DATA_BLOCK DB 3


STRUCT
    D_0 : word := W#16#0;
    D_1 : word := W#16#0;
    D_2 : word := W#16#0;
    D_3 : word := W#16#0;
    D_4 : word := W#16#0;
    D_5 : word := W#16#0;
    D_6 : word := W#16#0;
    D_7 : word := W#16#0;
    D_8 : word := W#16#0;
    D_9 : word := W#16#3;
    D_10 : word := W#16#0;
    D_11 : word := W#16#200;
    D_12 : word := W#16#0;
    D_13 : word := W#16#4000;
    D_14 : word := W#16#0;
    D_15 : word := W#16#4000;
    D_16 : word := W#16#0;
    D_17 : word := W#16#200;
    D_18 : word := W#16#0;
    D_19 : word := W#16#200;
    D_20 : word := W#16#0;
    D_21 : word := W#16#200;
    D_22 : word := W#16#0;
    D_23 : word := W#16#200;
    D_24 : word := W#16#0;
    D_25 : word := W#16#200;
    D_26 : word := W#16#0;
    D_27 : word := W#16#200;
    D_28 : word := W#16#0;
    D_29 : word := W#16#200;
    D_30 : word := W#16#0;
    D_31 : word := W#16#200;
    D_32 : word := W#16#0;
  END_STRUCT
BEGIN

END_DATA_BLOCK

DATA_BLOCK DB 9


STRUCT
    D_0 : word := W#16#0;
    D_1 : word := W#16#0;
    D_2 : word := W#16#0;
    D_3 : word := W#16#0;
    D_4 : word := W#16#0;
    D_5 : word := W#16#0;
    D_6 : word := W#16#0;
    D_7 : word := W#16#0;
    D_8 : word := W#16#0;
    D_9 : word := W#16#0;
    D_10 : word := W#16#508;
    D_11 : word := W#16#2C00;
    D_12 : word := W#16#0;
    D_13 : word := W#16#F;
    D_14 : word := W#16#112E;
    D_15 : word := W#16#0;
  END_STRUCT
BEGIN

END_DATA_BLOCK

DATA_BLOCK DB 94


STRUCT
    D_0 : word := W#16#0;
    D_1 : word := W#16#25;
    D_2 : word := W#16#12;
    D_3 : word := W#16#200;
    D_4 : word := W#16#100;
    D_5 : word := W#16#100;
    D_6 : word := W#16#78;
    D_7 : word := W#16#3018;
    D_8 : word := W#16#2060;
    D_9 : word := W#16#0;
    D_10 : word := W#16#0;
    D_11 : word := W#16#0;
    D_12 : word := W#16#0;
    D_13 : word := W#16#0;
    D_14 : word := W#16#0;
    D_15 : word := W#16#0;
    D_16 : word := W#16#0;
    D_17 : word := W#16#2010;
    D_18 : word := W#16#2030;
    D_19 : word := W#16#2010;
    D_20 : word := W#16#1050;
    D_21 : word := W#16#2020;
    D_22 : word := W#16#2020;
    D_23 : word := W#16#2010;
    D_24 : word := W#16#2060;
    D_25 : word := W#16#2300;
    D_26 : word := W#16#2010;
    D_27 : word := W#16#2020;
    D_28 : word := W#16#2005;
    D_29 : word := W#16#2030;
    D_30 : word := W#16#2008;
    D_31 : word := W#16#2300;
    D_32 : word := W#16#1020;
    D_33 : word := W#16#1020;
    D_34 : word := W#16#2008;
    D_35 : word := W#16#2300;
    D_36 : word := W#16#2008;
    D_37 : word := W#16#2025;
    D_38 : word := W#16#2015;
    D_39 : word := W#16#2015;
    D_40 : word := W#16#2300;
    D_41 : word := W#16#1050;
    D_42 : word := W#16#1050;
    D_43 : word := W#16#1050;
    D_44 : word := W#16#2020;
    D_45 : word := W#16#2008;
    D_46 : word := W#16#2300;
    D_47 : word := W#16#2010;
    D_48 : word := W#16#2300;
    D_49 : word := W#16#2030;
    D_50 : word := W#16#2010;
    D_51 : word := W#16#2030;
    D_52 : word := W#16#2010;
    D_53 : word := W#16#2030;
    D_54 : word := W#16#1020;
    D_55 : word := W#16#1020;
    D_56 : word := W#16#1020;
    D_57 : word := W#16#1020;
    D_58 : word := W#16#1020;
    D_59 : word := W#16#1020;
    D_60 : word := W#16#3180;
    D_61 : word := W#16#2300;
    D_62 : word := W#16#2300;
    D_63 : word := W#16#1050;
    D_64 : word := W#16#1150;
    D_65 : word := W#16#2010;
    D_66 : word := W#16#2002;
    D_67 : word := W#16#2002;
    D_68 : word := W#16#2002;
    D_69 : word := W#16#2030;
    D_70 : word := W#16#2030;
    D_71 : word := W#16#2020;
    D_72 : word := W#16#2020;
    D_73 : word := W#16#2020;
    D_74 : word := W#16#2045;
    D_75 : word := W#16#2030;
    D_76 : word := W#16#2030;
    D_77 : word := W#16#2005;
    D_78 : word := W#16#2005;
    D_79 : word := W#16#2005;
    D_80 : word := W#16#2005;
    D_81 : word := W#16#2120;
    D_82 : word := W#16#2010;
    D_83 : word := W#16#2010;
    D_84 : word := W#16#2009;
    D_85 : word := W#16#2005;
    D_86 : word := W#16#2005;
    D_87 : word := W#16#2010;
    D_88 : word := W#16#2300;
    D_89 : word := W#16#0;
    D_90 : word := W#16#2180;
    D_91 : word := W#16#2180;
    D_92 : word := W#16#3030;
    D_93 : word := W#16#2015;
    D_94 : word := W#16#2120;
    D_95 : word := W#16#2300;
    D_96 : word := W#16#2420;
    D_97 : word := W#16#2420;
    D_98 : word := W#16#2300;
    D_99 : word := W#16#1010;
    D_100 : word := W#16#1010;
    D_101 : word := W#16#2060;
    D_102 : word := W#16#2300;
    D_103 : word := W#16#2060;
    D_104 : word := W#16#1020;
    D_105 : word := W#16#1020;
    D_106 : word := W#16#1010;
    D_107 : word := W#16#2060;
    D_108 : word := W#16#2045;
    D_109 : word := W#16#0;
    D_110 : word := W#16#0;
    D_111 : word := W#16#1010;
    D_112 : word := W#16#1020;
    D_113 : word := W#16#0;
    D_114 : word := W#16#0;
    D_115 : word := W#16#0;
    D_116 : word := W#16#0;
    D_117 : word := W#16#0;
    D_118 : word := W#16#0;
    D_119 : word := W#16#0;
    D_120 : word := W#16#0;
    D_121 : word := W#16#0;
    D_122 : word := W#16#0;
    D_123 : word := W#16#0;
    D_124 : word := W#16#0;
    D_125 : word := W#16#0;
    D_126 : word := W#16#0;
    D_127 : word := W#16#0;
    D_128 : word := W#16#0;
    D_129 : word := W#16#2002;
    D_130 : word := W#16#2003;
    D_131 : word := W#16#0;
    D_132 : word := W#16#0;
    D_133 : word := W#16#0;
  END_STRUCT
BEGIN

END_DATA_BLOCK

DATA_BLOCK DB 99


STRUCT
    D_0 : word := W#16#0;
    D_1 : word := W#16#0;
    D_2 : word := W#16#3;
    D_3 : word := W#16#6;
    D_4 : word := W#16#2;
    D_5 : word := W#16#C;
    D_6 : word := W#16#6;
    D_7 : word := W#16#6;
    D_8 : word := W#16#6;
    D_9 : word := W#16#6;
    D_10 : word := W#16#6;
    D_11 : word := W#16#6;
    D_12 : word := W#16#6;
    D_13 : word := W#16#6;
    D_14 : word := W#16#6;
    D_15 : word := W#16#6;
    D_16 : word := W#16#0;
    D_17 : word := W#16#A6;
    D_18 : word := W#16#53;
    D_19 : word := W#16#1F4;
    D_20 : word := W#16#0;
  END_STRUCT
BEGIN

END_DATA_BLOCK

DATA_BLOCK DB 100


STRUCT
    D_0 : word := W#16#0;
    D_1 : word := W#16#5A;
    D_2 : word := W#16#0;
    D_3 : word := W#16#0;
    D_4 : word := W#16#0;
    D_5 : word := W#16#0;
    D_6 : word := W#16#0;
    D_7 : word := W#16#0;
    D_8 : word := W#16#0;
    D_9 : word := W#16#0;
    D_10 : word := W#16#8001;
    D_11 : word := W#16#8000;
    D_12 : word := W#16#8002;
    D_13 : word := W#16#8100;
    D_14 : word := W#16#8104;
    D_15 : word := W#16#8104;
    D_16 : word := W#16#8001;
    D_17 : word := W#16#8104;
    D_18 : word := W#16#8000;
    D_19 : word := W#16#8004;
    D_20 : word := W#16#8104;
    D_21 : word := W#16#8104;
    D_22 : word := W#16#8100;
    D_23 : word := W#16#8104;
    D_24 : word := W#16#8900;
    D_25 : word := W#16#8104;
    D_26 : word := W#16#8000;
    D_27 : word := W#16#8004;
    D_28 : word := W#16#8104;
    D_29 : word := W#16#8104;
    D_30 : word := W#16#8100;
    D_31 : word := W#16#8104;
    D_32 : word := W#16#8106;
    D_33 : word := W#16#8104;
    D_34 : word := W#16#8100;
    D_35 : word := W#16#8104;
    D_36 : word := W#16#8900;
    D_37 : word := W#16#8104;
    D_38 : word := W#16#100;
    D_39 : word := W#16#100;
    D_40 : word := W#16#100;
    D_41 : word := W#16#100;
    D_42 : word := W#16#8004;
    D_43 : word := W#16#8004;
    D_44 : word := W#16#4129;
    D_45 : word := W#16#412D;
    D_46 : word := W#16#8100;
    D_47 : word := W#16#8801;
    D_48 : word := W#16#8004;
    D_49 : word := W#16#8000;
    D_50 : word := W#16#8000;
    D_51 : word := W#16#815A;
    D_52 : word := W#16#8000;
    D_53 : word := W#16#8000;
    D_54 : word := W#16#8801;
    D_55 : word := W#16#8100;
    D_56 : word := W#16#8002;
    D_57 : word := W#16#8002;
    D_58 : word := W#16#8001;
    D_59 : word := W#16#8004;
    D_60 : word := W#16#8000;
    D_61 : word := W#16#8104;
    D_62 : word := W#16#8002;
    D_63 : word := W#16#8001;
    D_64 : word := W#16#8000;
    D_65 : word := W#16#8000;
    D_66 : word := W#16#8004;
    D_67 : word := W#16#8100;
    D_68 : word := W#16#8104;
    D_69 : word := W#16#8102;
    D_70 : word := W#16#8100;
    D_71 : word := W#16#8100;
    D_72 : word := W#16#8000;
    D_73 : word := W#16#8000;
    D_74 : word := W#16#100;
    D_75 : word := W#16#8001;
    D_76 : word := W#16#100;
    D_77 : word := W#16#8002;
    D_78 : word := W#16#8000;
    D_79 : word := W#16#8000;
    D_80 : word := W#16#100;
    D_81 : word := W#16#8002;
    D_82 : word := W#16#8100;
    D_83 : word := W#16#8002;
    D_84 : word := W#16#8801;
    D_85 : word := W#16#8102;
    D_86 : word := W#16#8002;
    D_87 : word := W#16#8002;
    D_88 : word := W#16#8000;
    D_89 : word := W#16#8801;
    D_90 : word := W#16#100;
    D_91 : word := W#16#100;
    D_92 : word := W#16#100;
    D_93 : word := W#16#100;
    D_94 : word := W#16#100;
    D_95 : word := W#16#100;
    D_96 : word := W#16#100;
    D_97 : word := W#16#100;
    D_98 : word := W#16#100;
    D_99 : word := W#16#100;
    D_100 : word := W#16#0;
    D_101 : word := W#16#0;
    D_102 : word := W#16#0;
    D_103 : word := W#16#0;
    D_104 : word := W#16#0;
    D_105 : word := W#16#0;
    D_106 : word := W#16#0;
    D_107 : word := W#16#0;
    D_108 : word := W#16#0;
    D_109 : word := W#16#0;
    D_110 : word := W#16#F;
    D_111 : word := W#16#5;
    D_112 : word := W#16#5;
    D_113 : word := W#16#5;
    D_114 : word := W#16#5;
    D_115 : word := W#16#5;
    D_116 : word := W#16#F;
    D_117 : word := W#16#5;
    D_118 : word := W#16#5;
    D_119 : word := W#16#5;
    D_120 : word := W#16#5;
    D_121 : word := W#16#5;
    D_122 : word := W#16#5;
    D_123 : word := W#16#5;
    D_124 : word := W#16#5;
    D_125 : word := W#16#5;
    D_126 : word := W#16#5;
    D_127 : word := W#16#5;
    D_128 : word := W#16#5;
    D_129 : word := W#16#5;
    D_130 : word := W#16#5;
    D_131 : word := W#16#5;
    D_132 : word := W#16#5;
    D_133 : word := W#16#5;
    D_134 : word := W#16#5;
    D_135 : word := W#16#5;
    D_136 : word := W#16#5;
    D_137 : word := W#16#5;
    D_138 : word := W#16#5;
    D_139 : word := W#16#5;
    D_140 : word := W#16#5;
    D_141 : word := W#16#5;
    D_142 : word := W#16#5;
    D_143 : word := W#16#5;
    D_144 : word := W#16#0;
    D_145 : word := W#16#0;
    D_146 : word := W#16#5;
    D_147 : word := W#16#F;
    D_148 : word := W#16#5;
    D_149 : word := W#16#5;
    D_150 : word := W#16#5;
    D_151 : word := W#16#5;
    D_152 : word := W#16#5;
    D_153 : word := W#16#5;
    D_154 : word := W#16#F;
    D_155 : word := W#16#5;
    D_156 : word := W#16#5;
    D_157 : word := W#16#5;
    D_158 : word := W#16#F;
    D_159 : word := W#16#5;
    D_160 : word := W#16#5;
    D_161 : word := W#16#5;
    D_162 : word := W#16#5;
    D_163 : word := W#16#F;
    D_164 : word := W#16#5;
    D_165 : word := W#16#5;
    D_166 : word := W#16#5;
    D_167 : word := W#16#5;
    D_168 : word := W#16#5;
    D_169 : word := W#16#5;
    D_170 : word := W#16#5;
    D_171 : word := W#16#5;
    D_172 : word := W#16#5;
    D_173 : word := W#16#5;
    D_174 : word := W#16#5;
    D_175 : word := W#16#F;
    D_176 : word := W#16#5;
    D_177 : word := W#16#5;
    D_178 : word := W#16#5;
    D_179 : word := W#16#F;
    D_180 : word := W#16#5;
    D_181 : word := W#16#5;
    D_182 : word := W#16#5;
    D_183 : word := W#16#5;
    D_184 : word := W#16#F;
    D_185 : word := W#16#5;
    D_186 : word := W#16#5;
    D_187 : word := W#16#5;
    D_188 : word := W#16#5;
    D_189 : word := W#16#F;
    D_190 : word := W#16#5;
    D_191 : word := W#16#5;
    D_192 : word := W#16#5;
    D_193 : word := W#16#5;
    D_194 : word := W#16#5;
    D_195 : word := W#16#5;
    D_196 : word := W#16#5;
    D_197 : word := W#16#5;
    D_198 : word := W#16#5;
    D_199 : word := W#16#5;
    D_200 : word := W#16#0;
  END_STRUCT
BEGIN

END_DATA_BLOCK

DATA_BLOCK DB 108


STRUCT
    D_0 : word := W#16#0;
    D_1 : word := W#16#0;
    D_2 : word := W#16#0;
    D_3 : word := W#16#0;
    D_4 : word := W#16#0;
    D_5 : word := W#16#0;
    D_6 : word := W#16#0;
    D_7 : word := W#16#0;
    D_8 : word := W#16#0;
    D_9 : word := W#16#0;
    D_10 : word := W#16#300;
    D_11 : word := W#16#3;
    D_12 : word := W#16#404;
    D_13 : word := W#16#300;
    D_14 : word := W#16#303;
    D_15 : word := W#16#404;
    D_16 : word := W#16#400;
    D_17 : word := W#16#303;
    D_18 : word := W#16#303;
    D_19 : word := W#16#404;
    D_20 : word := W#16#400;
    D_21 : word := W#16#406;
    D_22 : word := W#16#300;
    D_23 : word := W#16#303;
    D_24 : word := W#16#0;
    D_25 : word := W#16#0;
    D_26 : word := W#16#303;
    D_27 : word := W#16#202;
    D_28 : word := W#16#0;
    D_29 : word := W#16#303;
    D_30 : word := W#16#5A03;
    D_31 : word := W#16#303;
    D_32 : word := W#16#300;
    D_33 : word := W#16#303;
    D_34 : word := W#16#300;
    D_35 : word := W#16#303;
    D_36 : word := W#16#3;
    D_37 : word := W#16#303;
    D_38 : word := W#16#303;
    D_39 : word := W#16#303;
    D_40 : word := W#16#303;
    D_41 : word := W#16#303;
    D_42 : word := W#16#0;
    D_43 : word := W#16#300;
    D_44 : word := W#16#303;
    D_45 : word := W#16#300;
    D_46 : word := W#16#303;
    D_47 : word := W#16#300;
    D_48 : word := W#16#303;
    D_49 : word := W#16#3;
    D_50 : word := W#16#0;
    D_51 : word := W#16#0;
    D_52 : word := W#16#0;
    D_53 : word := W#16#0;
    D_54 : word := W#16#0;
    D_55 : word := W#16#0;
    D_56 : word := W#16#0;
    D_57 : word := W#16#0;
    D_58 : word := W#16#0;
    D_59 : word := W#16#0;
    D_60 : word := W#16#0;
  END_STRUCT
BEGIN

END_DATA_BLOCK

DATA_BLOCK DB 110


STRUCT
    D_0 : word := W#16#0;
    D_1 : word := W#16#3A;
    D_2 : word := W#16#0;
    D_3 : word := W#16#0;
    D_4 : word := W#16#0;
    D_5 : word := W#16#0;
    D_6 : word := W#16#0;
    D_7 : word := W#16#0;
    D_8 : word := W#16#0;
    D_9 : word := W#16#0;
    D_10 : word := W#16#8128;
    D_11 : word := W#16#8128;
    D_12 : word := W#16#8128;
    D_13 : word := W#16#8128;
    D_14 : word := W#16#404A;
    D_15 : word := W#16#484A;
    D_16 : word := W#16#102;
    D_17 : word := W#16#C828;
    D_18 : word := W#16#C128;
    D_19 : word := W#16#C128;
    D_20 : word := W#16#100;
    D_21 : word := W#16#802;
    D_22 : word := W#16#802;
    D_23 : word := W#16#C118;
    D_24 : word := W#16#101;
    D_25 : word := W#16#8128;
    D_26 : word := W#16#8128;
    D_27 : word := W#16#8128;
    D_28 : word := W#16#100;
    D_29 : word := W#16#100;
    D_30 : word := W#16#100;
    D_31 : word := W#16#100;
    D_32 : word := W#16#100;
    D_33 : word := W#16#100;
    D_34 : word := W#16#100;
    D_35 : word := W#16#100;
    D_36 : word := W#16#100;
    D_37 : word := W#16#100;
    D_38 : word := W#16#100;
    D_39 : word := W#16#100;
    D_40 : word := W#16#102;
    D_41 : word := W#16#102;
    D_42 : word := W#16#102;
    D_43 : word := W#16#102;
    D_44 : word := W#16#102;
    D_45 : word := W#16#102;
    D_46 : word := W#16#101;
    D_47 : word := W#16#102;
    D_48 : word := W#16#100;
    D_49 : word := W#16#100;
    D_50 : word := W#16#100;
    D_51 : word := W#16#100;
    D_52 : word := W#16#100;
    D_53 : word := W#16#100;
    D_54 : word := W#16#100;
    D_55 : word := W#16#100;
    D_56 : word := W#16#100;
    D_57 : word := W#16#102;
    D_58 : word := W#16#100;
    D_59 : word := W#16#100;
    D_60 : word := W#16#100;
    D_61 : word := W#16#100;
    D_62 : word := W#16#100;
    D_63 : word := W#16#100;
    D_64 : word := W#16#100;
    D_65 : word := W#16#100;
    D_66 : word := W#16#100;
    D_67 : word := W#16#100;
    D_68 : word := W#16#100;
    D_69 : word := W#16#100;
    D_70 : word := W#16#0;
    D_71 : word := W#16#0;
    D_72 : word := W#16#0;
    D_73 : word := W#16#0;
    D_74 : word := W#16#0;
    D_75 : word := W#16#0;
    D_76 : word := W#16#0;
    D_77 : word := W#16#0;
    D_78 : word := W#16#0;
    D_79 : word := W#16#0;
    D_80 : word := W#16#0;
    D_81 : word := W#16#0;
    D_82 : word := W#16#0;
    D_83 : word := W#16#0;
    D_84 : word := W#16#0;
    D_85 : word := W#16#0;
    D_86 : word := W#16#0;
    D_87 : word := W#16#0;
    D_88 : word := W#16#0;
    D_89 : word := W#16#0;
    D_90 : word := W#16#0;
    D_91 : word := W#16#0;
    D_92 : word := W#16#0;
    D_93 : word := W#16#0;
    D_94 : word := W#16#0;
    D_95 : word := W#16#0;
    D_96 : word := W#16#0;
    D_97 : word := W#16#0;
    D_98 : word := W#16#0;
    D_99 : word := W#16#0;
    D_100 : word := W#16#0;
    D_101 : word := W#16#0;
    D_102 : word := W#16#0;
    D_103 : word := W#16#0;
    D_104 : word := W#16#0;
    D_105 : word := W#16#0;
    D_106 : word := W#16#0;
    D_107 : word := W#16#0;
    D_108 : word := W#16#0;
    D_109 : word := W#16#0;
    D_110 : word := W#16#14;
    D_111 : word := W#16#14;
    D_112 : word := W#16#14;
    D_113 : word := W#16#14;
    D_114 : word := W#16#14;
    D_115 : word := W#16#14;
    D_116 : word := W#16#14;
    D_117 : word := W#16#0;
    D_118 : word := W#16#0;
    D_119 : word := W#16#0;
    D_120 : word := W#16#14;
    D_121 : word := W#16#14;
    D_122 : word := W#16#14;
    D_123 : word := W#16#0;
    D_124 : word := W#16#14;
    D_125 : word := W#16#14;
    D_126 : word := W#16#14;
    D_127 : word := W#16#14;
    D_128 : word := W#16#14;
    D_129 : word := W#16#14;
    D_130 : word := W#16#14;
    D_131 : word := W#16#14;
    D_132 : word := W#16#14;
    D_133 : word := W#16#14;
    D_134 : word := W#16#14;
    D_135 : word := W#16#14;
    D_136 : word := W#16#14;
    D_137 : word := W#16#14;
    D_138 : word := W#16#14;
    D_139 : word := W#16#14;
    D_140 : word := W#16#14;
    D_141 : word := W#16#14;
    D_142 : word := W#16#14;
    D_143 : word := W#16#14;
    D_144 : word := W#16#14;
    D_145 : word := W#16#14;
    D_146 : word := W#16#14;
    D_147 : word := W#16#14;
    D_148 : word := W#16#14;
    D_149 : word := W#16#14;
    D_150 : word := W#16#14;
    D_151 : word := W#16#14;
    D_152 : word := W#16#14;
    D_153 : word := W#16#14;
    D_154 : word := W#16#14;
    D_155 : word := W#16#14;
    D_156 : word := W#16#14;
    D_157 : word := W#16#14;
    D_158 : word := W#16#14;
    D_159 : word := W#16#14;
    D_160 : word := W#16#14;
    D_161 : word := W#16#14;
    D_162 : word := W#16#14;
    D_163 : word := W#16#14;
    D_164 : word := W#16#14;
    D_165 : word := W#16#14;
    D_166 : word := W#16#14;
    D_167 : word := W#16#14;
    D_168 : word := W#16#14;
    D_169 : word := W#16#14;
    D_170 : word := W#16#14;
    D_171 : word := W#16#14;
    D_172 : word := W#16#14;
    D_173 : word := W#16#14;
    D_174 : word := W#16#14;
    D_175 : word := W#16#14;
    D_176 : word := W#16#14;
    D_177 : word := W#16#14;
    D_178 : word := W#16#14;
    D_179 : word := W#16#14;
    D_180 : word := W#16#14;
    D_181 : word := W#16#14;
    D_182 : word := W#16#14;
    D_183 : word := W#16#14;
    D_184 : word := W#16#14;
    D_185 : word := W#16#14;
    D_186 : word := W#16#14;
    D_187 : word := W#16#14;
    D_188 : word := W#16#14;
    D_189 : word := W#16#14;
    D_190 : word := W#16#14;
    D_191 : word := W#16#14;
    D_192 : word := W#16#14;
    D_193 : word := W#16#14;
    D_194 : word := W#16#14;
    D_195 : word := W#16#14;
    D_196 : word := W#16#14;
    D_197 : word := W#16#14;
    D_198 : word := W#16#14;
    D_199 : word := W#16#14;
    D_200 : word := W#16#0;
  END_STRUCT
BEGIN

END_DATA_BLOCK

DATA_BLOCK DB 118


STRUCT
    D_0 : word := W#16#0;
    D_1 : word := W#16#0;
    D_2 : word := W#16#0;
    D_3 : word := W#16#0;
    D_4 : word := W#16#0;
    D_5 : word := W#16#0;
    D_6 : word := W#16#0;
    D_7 : word := W#16#0;
    D_8 : word := W#16#0;
    D_9 : word := W#16#0;
    D_10 : word := W#16#2828;
    D_11 : word := W#16#0;
    D_12 : word := W#16#202;
    D_13 : word := W#16#200;
    D_14 : word := W#16#202;
    D_15 : word := W#16#300;
    D_16 : word := W#16#203;
    D_17 : word := W#16#2801;
    D_18 : word := W#16#2828;
    D_19 : word := W#16#0;
    D_20 : word := W#16#0;
    D_21 : word := W#16#0;
    D_22 : word := W#16#0;
    D_23 : word := W#16#0;
    D_24 : word := W#16#0;
    D_25 : word := W#16#202;
    D_26 : word := W#16#202;
    D_27 : word := W#16#202;
    D_28 : word := W#16#205;
    D_29 : word := W#16#0;
    D_30 : word := W#16#0;
    D_31 : word := W#16#0;
    D_32 : word := W#16#0;
    D_33 : word := W#16#0;
    D_34 : word := W#16#0;
    D_35 : word := W#16#0;
    D_36 : word := W#16#0;
    D_37 : word := W#16#0;
    D_38 : word := W#16#0;
    D_39 : word := W#16#0;
    D_40 : word := W#16#0;
    D_41 : word := W#16#0;
    D_42 : word := W#16#0;
    D_43 : word := W#16#0;
    D_44 : word := W#16#0;
    D_45 : word := W#16#0;
    D_46 : word := W#16#0;
    D_47 : word := W#16#0;
    D_48 : word := W#16#0;
    D_49 : word := W#16#0;
    D_50 : word := W#16#0;
    D_51 : word := W#16#0;
    D_52 : word := W#16#0;
    D_53 : word := W#16#0;
    D_54 : word := W#16#0;
    D_55 : word := W#16#0;
    D_56 : word := W#16#0;
    D_57 : word := W#16#0;
    D_58 : word := W#16#0;
    D_59 : word := W#16#0;
    D_60 : word := W#16#0;
  END_STRUCT
BEGIN

END_DATA_BLOCK

DATA_BLOCK DB 120


STRUCT
    D_0 : word := W#16#0;
    D_1 : word := W#16#0;
    D_2 : word := W#16#0;
    D_3 : word := W#16#0;
    D_4 : word := W#16#0;
    D_5 : word := W#16#0;
    D_6 : word := W#16#0;
    D_7 : word := W#16#0;
    D_8 : word := W#16#0;
    D_9 : word := W#16#0;
    D_10 : word := W#16#5FC9;
    D_11 : word := W#16#40CF;
    D_12 : word := W#16#71D7;
    D_13 : word := W#16#80;
    D_14 : word := W#16#0;
    D_15 : word := W#16#8213;
    D_16 : word := W#16#0;
    D_17 : word := W#16#416C;
    D_18 : word := W#16#8;
    D_19 : word := W#16#2000;
    D_20 : word := W#16#C;
    D_21 : word := W#16#8018;
    D_22 : word := W#16#0;
    D_23 : word := W#16#7002;
    D_24 : word := W#16#9002;
    D_25 : word := W#16#3E14;
    D_26 : word := W#16#0;
    D_27 : word := W#16#200;
    D_28 : word := W#16#0;
    D_29 : word := W#16#4000;
    D_30 : word := W#16#0;
    D_31 : word := W#16#4000;
    D_32 : word := W#16#0;
    D_33 : word := W#16#0;
    D_34 : word := W#16#0;
    D_35 : word := W#16#0;
    D_36 : word := W#16#0;
    D_37 : word := W#16#0;
    D_38 : word := W#16#0;
    D_39 : word := W#16#0;
    D_40 : word := W#16#0;
    D_41 : word := W#16#0;
    D_42 : word := W#16#0;
    D_43 : word := W#16#0;
    D_44 : word := W#16#0;
    D_45 : word := W#16#0;
    D_46 : word := W#16#0;
    D_47 : word := W#16#0;
    D_48 : word := W#16#0;
    D_49 : word := W#16#0;
    D_50 : word := W#16#0;
    D_51 : word := W#16#0;
    D_52 : word := W#16#0;
    D_53 : word := W#16#0;
    D_54 : word := W#16#0;
    D_55 : word := W#16#0;
    D_56 : word := W#16#0;
    D_57 : word := W#16#0;
    D_58 : word := W#16#0;
    D_59 : word := W#16#0;
    D_60 : word := W#16#0;
    D_61 : word := W#16#0;
    D_62 : word := W#16#0;
    D_63 : word := W#16#0;
    D_64 : word := W#16#0;
    D_65 : word := W#16#0;
    D_66 : word := W#16#0;
    D_67 : word := W#16#0;
    D_68 : word := W#16#0;
    D_69 : word := W#16#0;
    D_70 : word := W#16#0;
    D_71 : word := W#16#0;
    D_72 : word := W#16#0;
    D_73 : word := W#16#0;
    D_74 : word := W#16#0;
    D_75 : word := W#16#0;
    D_76 : word := W#16#0;
    D_77 : word := W#16#0;
    D_78 : word := W#16#0;
    D_79 : word := W#16#0;
    D_80 : word := W#16#AA00;
    D_81 : word := W#16#0;
    D_82 : word := W#16#270;
    D_83 : word := W#16#2008;
    D_84 : word := W#16#2;
    D_85 : word := W#16#E83;
    D_86 : word := W#16#0;
    D_87 : word := W#16#8002;
    D_88 : word := W#16#1E2;
    D_89 : word := W#16#9;
    D_90 : word := W#16#600;
    D_91 : word := W#16#842E;
    D_92 : word := W#16#1801;
    D_93 : word := W#16#1800;
    D_94 : word := W#16#9B73;
    D_95 : word := W#16#0;
    D_96 : word := W#16#AA00;
    D_97 : word := W#16#0;
    D_98 : word := W#16#240C;
    D_99 : word := W#16#0;
    D_100 : word := W#16#0;
    D_101 : word := W#16#0;
    D_102 : word := W#16#0;
    D_103 : word := W#16#0;
    D_104 : word := W#16#0;
    D_105 : word := W#16#0;
    D_106 : word := W#16#0;
    D_107 : word := W#16#0;
    D_108 : word := W#16#0;
    D_109 : word := W#16#1;
    D_110 : word := W#16#1EEF;
    D_111 : word := W#16#FCFF;
    D_112 : word := W#16#FF0E;
    D_113 : word := W#16#0;
    D_114 : word := W#16#0;
    D_115 : word := W#16#0;
    D_116 : word := W#16#0;
    D_117 : word := W#16#0;
    D_118 : word := W#16#0;
    D_119 : word := W#16#0;
    D_120 : word := W#16#0;
    D_121 : word := W#16#0;
    D_122 : word := W#16#0;
    D_123 : word := W#16#0;
    D_124 : word := W#16#0;
    D_125 : word := W#16#0;
    D_126 : word := W#16#0;
    D_127 : word := W#16#0;
    D_128 : word := W#16#0;
    D_129 : word := W#16#0;
    D_130 : word := W#16#0;
    D_131 : word := W#16#0;
    D_132 : word := W#16#0;
    D_133 : word := W#16#0;
    D_134 : word := W#16#0;
    D_135 : word := W#16#0;
    D_136 : word := W#16#0;
    D_137 : word := W#16#0;
    D_138 : word := W#16#0;
    D_139 : word := W#16#0;
    D_140 : word := W#16#0;
    D_141 : word := W#16#0;
    D_142 : word := W#16#0;
    D_143 : word := W#16#0;
    D_144 : word := W#16#0;
    D_145 : word := W#16#0;
    D_146 : word := W#16#0;
    D_147 : word := W#16#0;
    D_148 : word := W#16#0;
    D_149 : word := W#16#0;
    D_150 : word := W#16#0;
    D_151 : word := W#16#0;
    D_152 : word := W#16#0;
    D_153 : word := W#16#0;
    D_154 : word := W#16#0;
  END_STRUCT
BEGIN

END_DATA_BLOCK

DATA_BLOCK DB 129


STRUCT
    D_0 : word := W#16#0;
    D_1 : word := W#16#0;
    D_2 : word := W#16#0;
    D_3 : word := W#16#0;
    D_4 : word := W#16#0;
    D_5 : word := W#16#0;
    D_6 : word := W#16#0;
    D_7 : word := W#16#0;
    D_8 : word := W#16#0;
    D_9 : word := W#16#0;
    D_10 : word := W#16#0;
    D_11 : word := W#16#0;
    D_12 : word := W#16#1048;
    D_13 : word := W#16#0;
    D_14 : word := W#16#0;
    D_15 : word := W#16#0;
  END_STRUCT
BEGIN

END_DATA_BLOCK

DATA_BLOCK DB 130


STRUCT
    D_0 : word := W#16#0;
    D_1 : word := W#16#0;
    D_2 : word := W#16#0;
    D_3 : word := W#16#0;
    D_4 : word := W#16#0;
    D_5 : word := W#16#0;
    D_6 : word := W#16#0;
    D_7 : word := W#16#0;
    D_8 : word := W#16#1E;
    D_9 : word := W#16#0;
    D_10 : word := W#16#1;
    D_11 : word := W#16#0;
    D_12 : word := W#16#89;
    D_13 : word := W#16#70E;
    D_14 : word := W#16#117;
    D_15 : word := W#16#617;
    D_16 : word := W#16#1;
    D_17 : word := W#16#610;
    D_18 : word := W#16#0;
    D_19 : word := W#16#862;
    D_20 : word := W#16#4;
    D_21 : word := W#16#1;
    D_22 : word := W#16#4;
    D_23 : word := W#16#1;
    D_24 : word := W#16#1;
    D_25 : word := W#16#1C;
    D_26 : word := W#16#23;
    D_27 : word := W#16#0;
    D_28 : word := W#16#0;
    D_29 : word := W#16#0;
    D_30 : word := W#16#0;
    D_31 : word := W#16#0;
    D_32 : word := W#16#441;
    D_33 : word := W#16#5C9;
    D_34 : word := W#16#33;
    D_35 : word := W#16#F;
    D_36 : word := W#16#7;
    D_37 : word := W#16#0;
    D_38 : word := W#16#0;
    D_39 : word := W#16#0;
    D_40 : word := W#16#0;
    D_41 : word := W#16#404;
    D_42 : word := W#16#19F;
    D_43 : word := W#16#0;
    D_44 : word := W#16#65A;
    D_45 : word := W#16#0;
    D_46 : word := W#16#572;
    D_47 : word := W#16#0;
    D_48 : word := W#16#1;
    D_49 : word := W#16#1;
    D_50 : word := W#16#75;
    D_51 : word := W#16#2;
    D_52 : word := W#16#1;
    D_53 : word := W#16#1;
    D_54 : word := W#16#1;
    D_55 : word := W#16#161;
    D_56 : word := W#16#1;
    D_57 : word := W#16#1;
    D_58 : word := W#16#1;
    D_59 : word := W#16#54D;
    D_60 : word := W#16#0;
    D_61 : word := W#16#5AC;
    D_62 : word := W#16#1;
    D_63 : word := W#16#1;
    D_64 : word := W#16#6AD;
    D_65 : word := W#16#956;
    D_66 : word := W#16#5E0;
    D_67 : word := W#16#1C2;
    D_68 : word := W#16#1E0;
    D_69 : word := W#16#194;
    D_70 : word := W#16#3FF;
    D_71 : word := W#16#2;
    D_72 : word := W#16#44F;
    D_73 : word := W#16#682;
    D_74 : word := W#16#2;
    D_75 : word := W#16#0;
    D_76 : word := W#16#0;
    D_77 : word := W#16#D3;
    D_78 : word := W#16#B70;
    D_79 : word := W#16#A29;
    D_80 : word := W#16#0;
    D_81 : word := W#16#0;
    D_82 : word := W#16#0;
    D_83 : word := W#16#4BC;
    D_84 : word := W#16#0;
    D_85 : word := W#16#0;
    D_86 : word := W#16#0;
    D_87 : word := W#16#0;
    D_88 : word := W#16#0;
    D_89 : word := W#16#0;
    D_90 : word := W#16#0;
    D_91 : word := W#16#0;
    D_92 : word := W#16#0;
    D_93 : word := W#16#0;
    D_94 : word := W#16#0;
    D_95 : word := W#16#7;
    D_96 : word := W#16#0;
    D_97 : word := W#16#0;
    D_98 : word := W#16#2B2;
    D_99 : word := W#16#0;
    D_100 : word := W#16#28D;
    D_101 : word := W#16#270;
    D_102 : word := W#16#0;
    D_103 : word := W#16#0;
    D_104 : word := W#16#0;
    D_105 : word := W#16#0;
    D_106 : word := W#16#2C3;
    D_107 : word := W#16#0;
    D_108 : word := W#16#0;
    D_109 : word := W#16#0;
    D_110 : word := W#16#0;
    D_111 : word := W#16#0;
    D_112 : word := W#16#0;
    D_113 : word := W#16#0;
    D_114 : word := W#16#308;
    D_115 : word := W#16#201;
    D_116 : word := W#16#60B;
    D_117 : word := W#16#281;
    D_118 : word := W#16#0;
    D_119 : word := W#16#0;
    D_120 : word := W#16#0;
    D_121 : word := W#16#117;
    D_122 : word := W#16#0;
    D_123 : word := W#16#0;
    D_124 : word := W#16#0;
    D_125 : word := W#16#0;
    D_126 : word := W#16#768;
    D_127 : word := W#16#0;
    D_128 : word := W#16#0;
    D_129 : word := W#16#0;
    D_130 : word := W#16#0;
    D_131 : word := W#16#0;
    D_132 : word := W#16#0;
    D_133 : word := W#16#0;
    D_134 : word := W#16#0;
    D_135 : word := W#16#0;
    D_136 : word := W#16#0;
    D_137 : word := W#16#0;
    D_138 : word := W#16#E;
    D_139 : word := W#16#6B;
    D_140 : word := W#16#14F;
    D_141 : word := W#16#27;
    D_142 : word := W#16#0;
    D_143 : word := W#16#D6;
    D_144 : word := W#16#0;
    D_145 : word := W#16#17;
    D_146 : word := W#16#120;
    D_147 : word := W#16#98;
    D_148 : word := W#16#A9;
    D_149 : word := W#16#131;
    D_150 : word := W#16#27;
    D_151 : word := W#16#228;
    D_152 : word := W#16#278;
    D_153 : word := W#16#23F;
    D_154 : word := W#16#E;
    D_155 : word := W#16#E;
    D_156 : word := W#16#0;
    D_157 : word := W#16#26;
    D_158 : word := W#16#0;
    D_159 : word := W#16#0;
    D_160 : word := W#16#0;
    D_161 : word := W#16#0;
    D_162 : word := W#16#2B;
    D_163 : word := W#16#1C;
    D_164 : word := W#16#27;
    D_165 : word := W#16#B;
    D_166 : word := W#16#23F;
    D_167 : word := W#16#98;
    D_168 : word := W#16#A;
    D_169 : word := W#16#27;
    D_170 : word := W#16#21;
    D_171 : word := W#16#22;
    D_172 : word := W#16#4B;
    D_173 : word := W#16#2C;
    D_174 : word := W#16#5A;
    D_175 : word := W#16#5C;
    D_176 : word := W#16#5B;
    D_177 : word := W#16#28;
    D_178 : word := W#16#BF;
    D_179 : word := W#16#3D;
    D_180 : word := W#16#E0;
    D_181 : word := W#16#70;
    D_182 : word := W#16#27;
    D_183 : word := W#16#27;
    D_184 : word := W#16#27;
    D_185 : word := W#16#27;
    D_186 : word := W#16#26;
    D_187 : word := W#16#26;
    D_188 : word := W#16#28;
    D_189 : word := W#16#27;
    D_190 : word := W#16#27;
    D_191 : word := W#16#27;
    D_192 : word := W#16#27;
    D_193 : word := W#16#27;
    D_194 : word := W#16#26;
    D_195 : word := W#16#27;
    D_196 : word := W#16#27;
    D_197 : word := W#16#28;
    D_198 : word := W#16#27;
    D_199 : word := W#16#27;
    D_200 : word := W#16#27;
    D_201 : word := W#16#27;
    D_202 : word := W#16#0;
    D_203 : word := W#16#0;
    D_204 : word := W#16#0;
    D_205 : word := W#16#0;
    D_206 : word := W#16#3A;
    D_207 : word := W#16#3A;
    D_208 : word := W#16#3A;
    D_209 : word := W#16#3A;
    D_210 : word := W#16#3A;
    D_211 : word := W#16#3A;
    D_212 : word := W#16#3A;
    D_213 : word := W#16#3A;
    D_214 : word := W#16#3A;
    D_215 : word := W#16#3A;
    D_216 : word := W#16#3A;
    D_217 : word := W#16#3A;
    D_218 : word := W#16#3A;
    D_219 : word := W#16#3A;
    D_220 : word := W#16#3A;
    D_221 : word := W#16#3A;
    D_222 : word := W#16#3A;
    D_223 : word := W#16#3A;
    D_224 : word := W#16#3A;
    D_225 : word := W#16#3A;
    D_226 : word := W#16#3A;
    D_227 : word := W#16#3A;
    D_228 : word := W#16#3A;
    D_229 : word := W#16#3A;
    D_230 : word := W#16#3A;
    D_231 : word := W#16#3A;
    D_232 : word := W#16#3A;
    D_233 : word := W#16#3A;
    D_234 : word := W#16#0;
    D_235 : word := W#16#0;
    D_236 : word := W#16#0;
    D_237 : word := W#16#0;
  END_STRUCT
BEGIN

END_DATA_BLOCK

DATA_BLOCK DB 131


STRUCT
    D_0 : word := W#16#0;
    D_1 : word := W#16#0;
    D_2 : word := W#16#0;
    D_3 : word := W#16#0;
    D_4 : word := W#16#0;
    D_5 : word := W#16#0;
    D_6 : word := W#16#0;
    D_7 : word := W#16#0;
    D_8 : word := W#16#0;
    D_9 : word := W#16#0;
    D_10 : word := W#16#CDFF;
    D_11 : word := W#16#CC33;
    D_12 : word := W#16#B34D;
    D_13 : word := W#16#CC1F;
    D_14 : word := W#16#E619;
    D_15 : word := W#16#E619;
    D_16 : word := W#16#FF00;
    D_17 : word := W#16#806E;
    D_18 : word := W#16#FF00;
    D_19 : word := W#16#FF00;
    D_20 : word := W#16#3300;
    D_21 : word := W#16#3300;
    D_22 : word := W#16#FF00;
    D_23 : word := W#16#FF00;
    D_24 : word := W#16#FF00;
    D_25 : word := W#16#FF77;
    D_26 : word := W#16#FF77;
    D_27 : word := W#16#FF77;
    D_28 : word := W#16#CD33;
    D_29 : word := W#16#FF00;
    D_30 : word := W#16#FF00;
    D_31 : word := W#16#FF00;
    D_32 : word := W#16#FF00;
    D_33 : word := W#16#806E;
    D_34 : word := W#16#C000;
    D_35 : word := W#16#FF00;
    D_36 : word := W#16#FF00;
    D_37 : word := W#16#FF00;
    D_38 : word := W#16#FF00;
    D_39 : word := W#16#FF11;
    D_40 : word := W#16#FF00;
    D_41 : word := W#16#CC00;
    D_42 : word := W#16#9A00;
    D_43 : word := W#16#E600;
    D_44 : word := W#16#806E;
    D_45 : word := W#16#806E;
    D_46 : word := W#16#806E;
    D_47 : word := W#16#FF00;
    D_48 : word := W#16#FF00;
    D_49 : word := W#16#FF00;
    D_50 : word := W#16#FF00;
    D_51 : word := W#16#FF00;
    D_52 : word := W#16#FF3D;
    D_53 : word := W#16#8000;
    D_54 : word := W#16#A000;
    D_55 : word := W#16#FF00;
    D_56 : word := W#16#FF00;
    D_57 : word := W#16#FF00;
    D_58 : word := W#16#806E;
    D_59 : word := W#16#806E;
    D_60 : word := W#16#806E;
    D_61 : word := W#16#FDF5;
    D_62 : word := W#16#4910;
    D_63 : word := W#16#FF00;
    D_64 : word := W#16#FF00;
    D_65 : word := W#16#FF00;
    D_66 : word := W#16#E633;
    D_67 : word := W#16#E640;
    D_68 : word := W#16#E640;
    D_69 : word := W#16#E640;
    D_70 : word := W#16#FF00;
    D_71 : word := W#16#9700;
    D_72 : word := W#16#806E;
    D_73 : word := W#16#806E;
    D_74 : word := W#16#FF00;
    D_75 : word := W#16#FF00;
    D_76 : word := W#16#E600;
    D_77 : word := W#16#FF00;
    D_78 : word := W#16#F40D;
    D_79 : word := W#16#FF00;
    D_80 : word := W#16#FF00;
    D_81 : word := W#16#FF8D;
    D_82 : word := W#16#8D00;
    D_83 : word := W#16#FF00;
    D_84 : word := W#16#FF00;
    D_85 : word := W#16#FF00;
    D_86 : word := W#16#F40D;
    D_87 : word := W#16#FF00;
    D_88 : word := W#16#FF00;
    D_89 : word := W#16#F40D;
    D_90 : word := W#16#FF00;
    D_91 : word := W#16#FF00;
    D_92 : word := W#16#F40D;
    D_93 : word := W#16#F40D;
    D_94 : word := W#16#FF00;
    D_95 : word := W#16#FF00;
    D_96 : word := W#16#FF00;
    D_97 : word := W#16#FF00;
    D_98 : word := W#16#FF00;
    D_99 : word := W#16#FF00;
    D_100 : word := W#16#A600;
    D_101 : word := W#16#FF00;
    D_102 : word := W#16#FF00;
    D_103 : word := W#16#FF00;
    D_104 : word := W#16#FF00;
    D_105 : word := W#16#FF00;
    D_106 : word := W#16#9200;
    D_107 : word := W#16#FF00;
    D_108 : word := W#16#FF00;
    D_109 : word := W#16#8400;
    D_110 : word := W#16#3300;
    D_111 : word := W#16#FF02;
    D_112 : word := W#16#FF00;
    D_113 : word := W#16#FF00;
    D_114 : word := W#16#33CD;
    D_115 : word := W#16#FF00;
    D_116 : word := W#16#FF00;
    D_117 : word := W#16#FF00;
    D_118 : word := W#16#FF00;
    D_119 : word := W#16#FF00;
    D_120 : word := W#16#E626;
    D_121 : word := W#16#FF00;
    D_122 : word := W#16#AA00;
    D_123 : word := W#16#BF00;
    D_124 : word := W#16#FF00;
    D_125 : word := W#16#5100;
    D_126 : word := W#16#5100;
    D_127 : word := W#16#FF00;
    D_128 : word := W#16#FF00;
    D_129 : word := W#16#FF00;
    D_130 : word := W#16#A600;
    D_131 : word := W#16#7700;
    D_132 : word := W#16#FF00;
    D_133 : word := W#16#FF00;
    D_134 : word := W#16#FF00;
    D_135 : word := W#16#FF00;
    D_136 : word := W#16#FF00;
    D_137 : word := W#16#FF00;
    D_138 : word := W#16#2D00;
    D_139 : word := W#16#2D00;
    D_140 : word := W#16#2D00;
    D_141 : word := W#16#A600;
    D_142 : word := W#16#2D00;
    D_143 : word := W#16#FF00;
    D_144 : word := W#16#FF00;
    D_145 : word := W#16#CB00;
    D_146 : word := W#16#FF00;
    D_147 : word := W#16#FF00;
    D_148 : word := W#16#CB00;
    D_149 : word := W#16#FF00;
    D_150 : word := W#16#FF00;
    D_151 : word := W#16#FF00;
    D_152 : word := W#16#3800;
    D_153 : word := W#16#9B00;
    D_154 : word := W#16#B00;
    D_155 : word := W#16#FF00;
    D_156 : word := W#16#FF00;
    D_157 : word := W#16#FF00;
    D_158 : word := W#16#FF00;
    D_159 : word := W#16#FF00;
    D_160 : word := W#16#6700;
    D_161 : word := W#16#6700;
    D_162 : word := W#16#C00;
    D_163 : word := W#16#C00;
    D_164 : word := W#16#A600;
    D_165 : word := W#16#C00;
    D_166 : word := W#16#FF00;
    D_167 : word := W#16#FF00;
    D_168 : word := W#16#C00;
    D_169 : word := W#16#C00;
    D_170 : word := W#16#C00;
    D_171 : word := W#16#C00;
    D_172 : word := W#16#C00;
    D_173 : word := W#16#C00;
    D_174 : word := W#16#FF00;
    D_175 : word := W#16#CF00;
    D_176 : word := W#16#FF00;
    D_177 : word := W#16#FF00;
    D_178 : word := W#16#FF00;
    D_179 : word := W#16#FF00;
    D_180 : word := W#16#FF00;
    D_181 : word := W#16#FF00;
    D_182 : word := W#16#FF00;
    D_183 : word := W#16#FF00;
    D_184 : word := W#16#FF00;
    D_185 : word := W#16#FF00;
    D_186 : word := W#16#FF00;
    D_187 : word := W#16#FF00;
    D_188 : word := W#16#FF00;
    D_189 : word := W#16#FF00;
    D_190 : word := W#16#FF00;
    D_191 : word := W#16#FF00;
    D_192 : word := W#16#FF00;
    D_193 : word := W#16#FF00;
    D_194 : word := W#16#FF00;
    D_195 : word := W#16#FF00;
    D_196 : word := W#16#FF00;
    D_197 : word := W#16#FF00;
    D_198 : word := W#16#FF00;
    D_199 : word := W#16#FF00;
    D_200 : word := W#16#FF00;
    D_201 : word := W#16#FF00;
    D_202 : word := W#16#0;
    D_203 : word := W#16#0;
    D_204 : word := W#16#0;
    D_205 : word := W#16#0;
    D_206 : word := W#16#0;
    D_207 : word := W#16#0;
  END_STRUCT
BEGIN

END_DATA_BLOCK

DATA_BLOCK DB 132


STRUCT
    D_0 : word := W#16#0;
    D_1 : word := W#16#0;
    D_2 : word := W#16#0;
    D_3 : word := W#16#0;
    D_4 : word := W#16#0;
    D_5 : word := W#16#0;
    D_6 : word := W#16#0;
    D_7 : word := W#16#0;
    D_8 : word := W#16#0;
    D_9 : word := W#16#0;
    D_10 : word := W#16#B340;
    D_11 : word := W#16#B34D;
    D_12 : word := W#16#9966;
    D_13 : word := W#16#B333;
    D_14 : word := W#16#E6D9;
    D_15 : word := W#16#E6D9;
    D_16 : word := W#16#E60D;
    D_17 : word := W#16#7C72;
    D_18 : word := W#16#FF00;
    D_19 : word := W#16#FF00;
    D_20 : word := W#16#FF00;
    D_21 : word := W#16#FF00;
    D_22 : word := W#16#FF00;
    D_23 : word := W#16#FF00;
    D_24 : word := W#16#FF00;
    D_25 : word := W#16#8000;
    D_26 : word := W#16#8000;
    D_27 : word := W#16#8000;
    D_28 : word := W#16#C040;
    D_29 : word := W#16#FF00;
    D_30 : word := W#16#FF00;
    D_31 : word := W#16#FF00;
    D_32 : word := W#16#FF00;
    D_33 : word := W#16#7C72;
    D_34 : word := W#16#BBFF;
    D_35 : word := W#16#FF00;
    D_36 : word := W#16#FF00;
    D_37 : word := W#16#FF00;
    D_38 : word := W#16#FF00;
    D_39 : word := W#16#F719;
    D_40 : word := W#16#FF00;
    D_41 : word := W#16#4D0D;
    D_42 : word := W#16#700;
    D_43 : word := W#16#CD00;
    D_44 : word := W#16#7C72;
    D_45 : word := W#16#7C72;
    D_46 : word := W#16#7C72;
    D_47 : word := W#16#FF00;
    D_48 : word := W#16#FF00;
    D_49 : word := W#16#FF00;
    D_50 : word := W#16#FF00;
    D_51 : word := W#16#FF00;
    D_52 : word := W#16#FF47;
    D_53 : word := W#16#7000;
    D_54 : word := W#16#9900;
    D_55 : word := W#16#FF00;
    D_56 : word := W#16#FF00;
    D_57 : word := W#16#3300;
    D_58 : word := W#16#7C72;
    D_59 : word := W#16#7C72;
    D_60 : word := W#16#7C72;
    D_61 : word := W#16#FBF8;
    D_62 : word := W#16#FF00;
    D_63 : word := W#16#FF00;
    D_64 : word := W#16#CC00;
    D_65 : word := W#16#FF00;
    D_66 : word := W#16#CD66;
    D_67 : word := W#16#CD00;
    D_68 : word := W#16#CD4D;
    D_69 : word := W#16#CD4D;
    D_70 : word := W#16#FF00;
    D_71 : word := W#16#FF00;
    D_72 : word := W#16#7C72;
    D_73 : word := W#16#7C72;
    D_74 : word := W#16#FF00;
    D_75 : word := W#16#FF00;
    D_76 : word := W#16#CD00;
    D_77 : word := W#16#FF00;
    D_78 : word := W#16#EE12;
    D_79 : word := W#16#FF00;
    D_80 : word := W#16#8000;
    D_81 : word := W#16#FF00;
    D_82 : word := W#16#8600;
    D_83 : word := W#16#B359;
    D_84 : word := W#16#FF00;
    D_85 : word := W#16#FF00;
    D_86 : word := W#16#EE12;
    D_87 : word := W#16#FF00;
    D_88 : word := W#16#FF00;
    D_89 : word := W#16#EE40;
    D_90 : word := W#16#FF00;
    D_91 : word := W#16#FF00;
    D_92 : word := W#16#EE12;
    D_93 : word := W#16#EE40;
    D_94 : word := W#16#FF00;
    D_95 : word := W#16#FF00;
    D_96 : word := W#16#FF00;
    D_97 : word := W#16#FF00;
    D_98 : word := W#16#FF00;
    D_99 : word := W#16#FF00;
    D_100 : word := W#16#A200;
    D_101 : word := W#16#FF00;
    D_102 : word := W#16#FF00;
    D_103 : word := W#16#FF00;
    D_104 : word := W#16#FF00;
    D_105 : word := W#16#FF00;
    D_106 : word := W#16#8A15;
    D_107 : word := W#16#F615;
    D_108 : word := W#16#F615;
    D_109 : word := W#16#7B15;
    D_110 : word := W#16#2E00;
    D_111 : word := W#16#FF00;
    D_112 : word := W#16#FF00;
    D_113 : word := W#16#FF00;
    D_114 : word := W#16#4DC0;
    D_115 : word := W#16#FF00;
    D_116 : word := W#16#FF00;
    D_117 : word := W#16#FF00;
    D_118 : word := W#16#FF00;
    D_119 : word := W#16#FF00;
    D_120 : word := W#16#D933;
    D_121 : word := W#16#FF00;
    D_122 : word := W#16#7800;
    D_123 : word := W#16#AA00;
    D_124 : word := W#16#FF00;
    D_125 : word := W#16#3D00;
    D_126 : word := W#16#3D00;
    D_127 : word := W#16#FF00;
    D_128 : word := W#16#FF00;
    D_129 : word := W#16#FF00;
    D_130 : word := W#16#F500;
    D_131 : word := W#16#6600;
    D_132 : word := W#16#FF00;
    D_133 : word := W#16#FF00;
    D_134 : word := W#16#FF00;
    D_135 : word := W#16#FF00;
    D_136 : word := W#16#FF00;
    D_137 : word := W#16#FF00;
    D_138 : word := W#16#2B1F;
    D_139 : word := W#16#2B1F;
    D_140 : word := W#16#2B1F;
    D_141 : word := W#16#2B1F;
    D_142 : word := W#16#2B1F;
    D_143 : word := W#16#FF00;
    D_144 : word := W#16#FF00;
    D_145 : word := W#16#C000;
    D_146 : word := W#16#FF00;
    D_147 : word := W#16#FF00;
    D_148 : word := W#16#C000;
    D_149 : word := W#16#FF00;
    D_150 : word := W#16#FF00;
    D_151 : word := W#16#FF00;
    D_152 : word := W#16#360C;
    D_153 : word := W#16#8634;
    D_154 : word := W#16#900;
    D_155 : word := W#16#1400;
    D_156 : word := W#16#1400;
    D_157 : word := W#16#1400;
    D_158 : word := W#16#1900;
    D_159 : word := W#16#1000;
    D_160 : word := W#16#5D00;
    D_161 : word := W#16#5D00;
    D_162 : word := W#16#700;
    D_163 : word := W#16#700;
    D_164 : word := W#16#800;
    D_165 : word := W#16#800;
    D_166 : word := W#16#FF00;
    D_167 : word := W#16#FF00;
    D_168 : word := W#16#700;
    D_169 : word := W#16#700;
    D_170 : word := W#16#700;
    D_171 : word := W#16#700;
    D_172 : word := W#16#700;
    D_173 : word := W#16#700;
    D_174 : word := W#16#FF00;
    D_175 : word := W#16#D00;
    D_176 : word := W#16#FF00;
    D_177 : word := W#16#FF00;
    D_178 : word := W#16#FF00;
    D_179 : word := W#16#FF00;
    D_180 : word := W#16#FF00;
    D_181 : word := W#16#FF00;
    D_182 : word := W#16#FF00;
    D_183 : word := W#16#FF00;
    D_184 : word := W#16#FF00;
    D_185 : word := W#16#FF00;
    D_186 : word := W#16#FF00;
    D_187 : word := W#16#FF00;
    D_188 : word := W#16#FF00;
    D_189 : word := W#16#FF00;
    D_190 : word := W#16#FF00;
    D_191 : word := W#16#FF00;
    D_192 : word := W#16#FF00;
    D_193 : word := W#16#FF00;
    D_194 : word := W#16#FF00;
    D_195 : word := W#16#FF00;
    D_196 : word := W#16#FF00;
    D_197 : word := W#16#FF00;
    D_198 : word := W#16#FF00;
    D_199 : word := W#16#FF00;
    D_200 : word := W#16#FF00;
    D_201 : word := W#16#FF00;
    D_202 : word := W#16#0;
    D_203 : word := W#16#0;
    D_204 : word := W#16#0;
    D_205 : word := W#16#0;
    D_206 : word := W#16#0;
  END_STRUCT
BEGIN

END_DATA_BLOCK

DATA_BLOCK DB 133


STRUCT
    D_0 : word := W#16#0;
    D_1 : word := W#16#0;
    D_2 : word := W#16#0;
    D_3 : word := W#16#0;
    D_4 : word := W#16#0;
    D_5 : word := W#16#0;
    D_6 : word := W#16#0;
    D_7 : word := W#16#0;
    D_8 : word := W#16#0;
    D_9 : word := W#16#0;
    D_10 : word := W#16#0;
    D_11 : word := W#16#1000;
    D_12 : word := W#16#0;
    D_13 : word := W#16#3;
    D_14 : word := W#16#0;
    D_15 : word := W#16#3;
    D_16 : word := W#16#0;
    D_17 : word := W#16#0;
    D_18 : word := W#16#0;
    D_19 : word := W#16#0;
    D_20 : word := W#16#0;
    D_21 : word := W#16#0;
    D_22 : word := W#16#400;
    D_23 : word := W#16#400;
    D_24 : word := W#16#9;
    D_25 : word := W#16#400;
    D_26 : word := W#16#400;
    D_27 : word := W#16#400;
    D_28 : word := W#16#162;
    D_29 : word := W#16#1F7;
    D_30 : word := W#16#12A;
    D_31 : word := W#16#0;
    D_32 : word := W#16#1;
    D_33 : word := W#16#1;
    D_34 : word := W#16#1;
    D_35 : word := W#16#1;
    D_36 : word := W#16#1;
    D_37 : word := W#16#1;
    D_38 : word := W#16#1AC;
    D_39 : word := W#16#400;
    D_40 : word := W#16#0;
    D_41 : word := W#16#0;
    D_42 : word := W#16#3;
    D_43 : word := W#16#7;
    D_44 : word := W#16#55;
    D_45 : word := W#16#0;
    D_46 : word := W#16#0;
    D_47 : word := W#16#0;
    D_48 : word := W#16#400;
    D_49 : word := W#16#400;
    D_50 : word := W#16#400;
    D_51 : word := W#16#400;
    D_52 : word := W#16#400;
    D_53 : word := W#16#400;
    D_54 : word := W#16#400;
    D_55 : word := W#16#400;
    D_56 : word := W#16#400;
    D_57 : word := W#16#400;
    D_58 : word := W#16#400;
    D_59 : word := W#16#400;
    D_60 : word := W#16#400;
    D_61 : word := W#16#400;
    D_62 : word := W#16#400;
    D_63 : word := W#16#400;
    D_64 : word := W#16#400;
    D_65 : word := W#16#400;
    D_66 : word := W#16#400;
    D_67 : word := W#16#400;
    D_68 : word := W#16#400;
    D_69 : word := W#16#400;
    D_70 : word := W#16#0;
    D_71 : word := W#16#0;
    D_72 : word := W#16#7FF;
    D_73 : word := W#16#7FF;
    D_74 : word := W#16#0;
    D_75 : word := W#16#0;
    D_76 : word := W#16#0;
    D_77 : word := W#16#0;
    D_78 : word := W#16#0;
    D_79 : word := W#16#0;
    D_80 : word := W#16#0;
    D_81 : word := W#16#0;
    D_82 : word := W#16#0;
    D_83 : word := W#16#0;
    D_84 : word := W#16#0;
    D_85 : word := W#16#0;
    D_86 : word := W#16#D5;
    D_87 : word := W#16#1F0;
    D_88 : word := W#16#17;
    D_89 : word := W#16#120;
    D_90 : word := W#16#346;
    D_91 : word := W#16#A8;
    D_92 : word := W#16#131;
    D_93 : word := W#16#27;
    D_94 : word := W#16#228;
    D_95 : word := W#16#7;
    D_96 : word := W#16#7;
    D_97 : word := W#16#7;
    D_98 : word := W#16#C;
    D_99 : word := W#16#53;
    D_100 : word := W#16#0;
    D_101 : word := W#16#0;
    D_102 : word := W#16#0;
    D_103 : word := W#16#0;
    D_104 : word := W#16#0;
    D_105 : word := W#16#0;
    D_106 : word := W#16#0;
    D_107 : word := W#16#0;
    D_108 : word := W#16#0;
    D_109 : word := W#16#0;
    D_110 : word := W#16#0;
  END_STRUCT
BEGIN

END_DATA_BLOCK

DATA_BLOCK DB 134


STRUCT
    D_0 : word := W#16#0;
    D_1 : word := W#16#0;
    D_2 : word := W#16#0;
    D_3 : word := W#16#0;
    D_4 : word := W#16#0;
    D_5 : word := W#16#0;
    D_6 : word := W#16#0;
    D_7 : word := W#16#0;
    D_8 : word := W#16#0;
    D_9 : word := W#16#0;
    D_10 : word := W#16#FF0D;
    D_11 : word := W#16#FF0D;
    D_12 : word := W#16#FF00;
    D_13 : word := W#16#9914;
    D_14 : word := W#16#9914;
    D_15 : word := W#16#FF00;
    D_16 : word := W#16#B333;
    D_17 : word := W#16#B333;
    D_18 : word := W#16#FF00;
    D_19 : word := W#16#FF00;
    D_20 : word := W#16#FF00;
    D_21 : word := W#16#FF00;
    D_22 : word := W#16#FF00;
    D_23 : word := W#16#FF00;
    D_24 : word := W#16#FF00;
    D_25 : word := W#16#FF00;
    D_26 : word := W#16#FF00;
    D_27 : word := W#16#FF00;
    D_28 : word := W#16#CE00;
    D_29 : word := W#16#CE00;
    D_30 : word := W#16#CE00;
    D_31 : word := W#16#FF00;
    D_32 : word := W#16#FF00;
    D_33 : word := W#16#FF00;
    D_34 : word := W#16#FF00;
    D_35 : word := W#16#FF00;
    D_36 : word := W#16#FF00;
    D_37 : word := W#16#FF00;
    D_38 : word := W#16#FF00;
    D_39 : word := W#16#FF00;
    D_40 : word := W#16#FF66;
    D_41 : word := W#16#6B20;
    D_42 : word := W#16#FF29;
    D_43 : word := W#16#FF00;
    D_44 : word := W#16#FF00;
    D_45 : word := W#16#FF00;
    D_46 : word := W#16#FF00;
    D_47 : word := W#16#FF00;
    D_48 : word := W#16#FF00;
    D_49 : word := W#16#FF00;
    D_50 : word := W#16#FF00;
    D_51 : word := W#16#FF00;
    D_52 : word := W#16#FF00;
    D_53 : word := W#16#FC00;
    D_54 : word := W#16#FF00;
    D_55 : word := W#16#FC00;
    D_56 : word := W#16#FF00;
    D_57 : word := W#16#FF00;
    D_58 : word := W#16#FF00;
    D_59 : word := W#16#FF00;
    D_60 : word := W#16#FF00;
    D_61 : word := W#16#FF00;
    D_62 : word := W#16#FF00;
    D_63 : word := W#16#FF00;
    D_64 : word := W#16#FF00;
    D_65 : word := W#16#FF00;
    D_66 : word := W#16#FF00;
    D_67 : word := W#16#FF00;
    D_68 : word := W#16#FF00;
    D_69 : word := W#16#FF00;
    D_70 : word := W#16#FF00;
    D_71 : word := W#16#FF00;
    D_72 : word := W#16#FF00;
    D_73 : word := W#16#FF00;
    D_74 : word := W#16#0;
    D_75 : word := W#16#0;
  END_STRUCT
BEGIN

END_DATA_BLOCK

DATA_BLOCK DB 135


STRUCT
    D_0 : word := W#16#0;
    D_1 : word := W#16#0;
    D_2 : word := W#16#0;
    D_3 : word := W#16#0;
    D_4 : word := W#16#0;
    D_5 : word := W#16#0;
    D_6 : word := W#16#0;
    D_7 : word := W#16#0;
    D_8 : word := W#16#0;
    D_9 : word := W#16#0;
    D_10 : word := W#16#FF59;
    D_11 : word := W#16#FF59;
    D_12 : word := W#16#FF00;
    D_13 : word := W#16#8E1F;
    D_14 : word := W#16#8E1F;
    D_15 : word := W#16#FF00;
    D_16 : word := W#16#9940;
    D_17 : word := W#16#9940;
    D_18 : word := W#16#FF00;
    D_19 : word := W#16#FF00;
    D_20 : word := W#16#FF00;
    D_21 : word := W#16#FF00;
    D_22 : word := W#16#FF00;
    D_23 : word := W#16#FF00;
    D_24 : word := W#16#FF00;
    D_25 : word := W#16#FF00;
    D_26 : word := W#16#FF00;
    D_27 : word := W#16#FF00;
    D_28 : word := W#16#C472;
    D_29 : word := W#16#C472;
    D_30 : word := W#16#C472;
    D_31 : word := W#16#FF00;
    D_32 : word := W#16#FF00;
    D_33 : word := W#16#FF00;
    D_34 : word := W#16#FF00;
    D_35 : word := W#16#FF00;
    D_36 : word := W#16#FF00;
    D_37 : word := W#16#FF00;
    D_38 : word := W#16#BA72;
    D_39 : word := W#16#FF00;
    D_40 : word := W#16#FF80;
    D_41 : word := W#16#502B;
    D_42 : word := W#16#FA33;
    D_43 : word := W#16#FF00;
    D_44 : word := W#16#FF00;
    D_45 : word := W#16#FF00;
    D_46 : word := W#16#FF00;
    D_47 : word := W#16#FF00;
    D_48 : word := W#16#FF00;
    D_49 : word := W#16#FF00;
    D_50 : word := W#16#FF00;
    D_51 : word := W#16#FF00;
    D_52 : word := W#16#FF00;
    D_53 : word := W#16#FF00;
    D_54 : word := W#16#FF00;
    D_55 : word := W#16#FF00;
    D_56 : word := W#16#FF00;
    D_57 : word := W#16#FF00;
    D_58 : word := W#16#FF00;
    D_59 : word := W#16#FF00;
    D_60 : word := W#16#FF00;
    D_61 : word := W#16#FF00;
    D_62 : word := W#16#FF00;
    D_63 : word := W#16#FF00;
    D_64 : word := W#16#FF00;
    D_65 : word := W#16#FF00;
    D_66 : word := W#16#FF00;
    D_67 : word := W#16#FF00;
    D_68 : word := W#16#FF00;
    D_69 : word := W#16#FF00;
    D_70 : word := W#16#FF00;
    D_71 : word := W#16#FF00;
    D_72 : word := W#16#FF00;
    D_73 : word := W#16#FF00;
    D_74 : word := W#16#0;
    D_75 : word := W#16#0;
  END_STRUCT
BEGIN

END_DATA_BLOCK

DATA_BLOCK DB 136


STRUCT
    D_0 : word := W#16#0;
    D_1 : word := W#16#0;
    D_2 : word := W#16#0;
    D_3 : word := W#16#0;
    D_4 : word := W#16#0;
    D_5 : word := W#16#0;
    D_6 : word := W#16#0;
    D_7 : word := W#16#0;
    D_8 : word := W#16#0;
    D_9 : word := W#16#0;
    D_10 : word := W#16#C333;
    D_11 : word := W#16#C222;
    D_12 : word := W#16#C0;
    D_13 : word := W#16#1000;
    D_14 : word := W#16#311;
    D_15 : word := W#16#C000;
    D_16 : word := W#16#2;
    D_17 : word := W#16#4030;
    D_18 : word := W#16#3C04;
    D_19 : word := W#16#C;
    D_20 : word := W#16#300;
    D_21 : word := W#16#0;
    D_22 : word := W#16#33C3;
    D_23 : word := W#16#C401;
    D_24 : word := W#16#3310;
    D_25 : word := W#16#CC00;
    D_26 : word := W#16#0;
    D_27 : word := W#16#10CC;
    D_28 : word := W#16#0;
    D_29 : word := W#16#3003;
    D_30 : word := W#16#3300;
    D_31 : word := W#16#0;
    D_32 : word := W#16#0;
    D_33 : word := W#16#0;
    D_34 : word := W#16#2220;
    D_35 : word := W#16#10;
    D_36 : word := W#16#F;
    D_37 : word := W#16#300;
    D_38 : word := W#16#0;
    D_39 : word := W#16#0;
    D_40 : word := W#16#0;
    D_41 : word := W#16#0;
    D_42 : word := W#16#2C22;
    D_43 : word := W#16#2;
    D_44 : word := W#16#0;
    D_45 : word := W#16#C00;
    D_46 : word := W#16#0;
    D_47 : word := W#16#0;
    D_48 : word := W#16#0;
    D_49 : word := W#16#0;
    D_50 : word := W#16#400;
    D_51 : word := W#16#0;
    D_52 : word := W#16#0;
    D_53 : word := W#16#0;
    D_54 : word := W#16#0;
    D_55 : word := W#16#0;
    D_56 : word := W#16#0;
    D_57 : word := W#16#0;
    D_58 : word := W#16#30C3;
    D_59 : word := W#16#3303;
    D_60 : word := W#16#0;
    D_61 : word := W#16#0;
    D_62 : word := W#16#2C00;
    D_63 : word := W#16#2;
    D_64 : word := W#16#0;
    D_65 : word := W#16#330C;
    D_66 : word := W#16#3;
    D_67 : word := W#16#0;
    D_68 : word := W#16#0;
    D_69 : word := W#16#0;
    D_70 : word := W#16#0;
    D_71 : word := W#16#0;
    D_72 : word := W#16#0;
    D_73 : word := W#16#CC00;
    D_74 : word := W#16#0;
    D_75 : word := W#16#0;
    D_76 : word := W#16#3033;
    D_77 : word := W#16#3303;
    D_78 : word := W#16#0;
    D_79 : word := W#16#0;
    D_80 : word := W#16#2200;
    D_81 : word := W#16#2;
    D_82 : word := W#16#0;
    D_83 : word := W#16#3302;
    D_84 : word := W#16#3;
    D_85 : word := W#16#0;
    D_86 : word := W#16#0;
    D_87 : word := W#16#0;
    D_88 : word := W#16#0;
    D_89 : word := W#16#0;
    D_90 : word := W#16#0;
    D_91 : word := W#16#CC00;
    D_92 : word := W#16#0;
    D_93 : word := W#16#0;
  END_STRUCT
BEGIN

END_DATA_BLOCK

DATA_BLOCK DB 138


STRUCT
    D_0 : word := W#16#0;
    D_1 : word := W#16#0;
    D_2 : word := W#16#0;
    D_3 : word := W#16#0;
    D_4 : word := W#16#0;
    D_5 : word := W#16#0;
    D_6 : word := W#16#0;
    D_7 : word := W#16#0;
    D_8 : word := W#16#0;
    D_9 : word := W#16#0;
    D_10 : word := W#16#1DD;
    D_11 : word := W#16#0;
    D_12 : word := W#16#49A;
    D_13 : word := W#16#3CC;
    D_14 : word := W#16#2A3;
    D_15 : word := W#16#370;
    D_16 : word := W#16#2D7;
    D_17 : word := W#16#200;
    D_18 : word := W#16#2A0;
    D_19 : word := W#16#EA;
    D_20 : word := W#16#124;
    D_21 : word := W#16#800;
    D_22 : word := W#16#0;
    D_23 : word := W#16#5D4;
    D_24 : word := W#16#507;
    D_25 : word := W#16#2CF;
    D_26 : word := W#16#8F;
    D_27 : word := W#16#8F;
    D_28 : word := W#16#D0;
    D_29 : word := W#16#798;
    D_30 : word := W#16#19;
    D_31 : word := W#16#0;
    D_32 : word := W#16#0;
    D_33 : word := W#16#0;
    D_34 : word := W#16#0;
    D_35 : word := W#16#0;
    D_36 : word := W#16#0;
    D_37 : word := W#16#0;
    D_38 : word := W#16#0;
    D_39 : word := W#16#0;
    D_40 : word := W#16#0;
    D_41 : word := W#16#0;
    D_42 : word := W#16#0;
    D_43 : word := W#16#0;
    D_44 : word := W#16#0;
    D_45 : word := W#16#0;
  END_STRUCT
BEGIN

END_DATA_BLOCK

DATA_BLOCK DB 140


STRUCT
    D_0 : word := W#16#0;
    D_1 : word := W#16#0;
    D_2 : word := W#16#0;
    D_3 : word := W#16#0;
    D_4 : word := W#16#0;
    D_5 : word := W#16#0;
    D_6 : word := W#16#0;
    D_7 : word := W#16#0;
    D_8 : word := W#16#0;
    D_9 : word := W#16#0;
    D_10 : word := W#16#0;
    D_11 : word := W#16#0;
    D_12 : word := W#16#0;
    D_13 : word := W#16#0;
    D_14 : word := W#16#1;
    D_15 : word := W#16#0;
    D_16 : word := W#16#0;
    D_17 : word := W#16#0;
    D_18 : word := W#16#0;
    D_19 : word := W#16#0;
    D_20 : word := W#16#0;
    D_21 : word := W#16#0;
    D_22 : word := W#16#0;
    D_23 : word := W#16#0;
    D_24 : word := W#16#1;
    D_25 : word := W#16#0;
    D_26 : word := W#16#0;
    D_27 : word := W#16#0;
    D_28 : word := W#16#0;
    D_29 : word := W#16#0;
    D_30 : word := W#16#FE58;
    D_31 : word := W#16#0;
    D_32 : word := W#16#0;
    D_33 : word := W#16#0;
    D_34 : word := W#16#1;
    D_35 : word := W#16#0;
    D_36 : word := W#16#0;
    D_37 : word := W#16#0;
    D_38 : word := W#16#0;
    D_39 : word := W#16#0;
    D_40 : word := W#16#FE58;
    D_41 : word := W#16#0;
    D_42 : word := W#16#0;
    D_43 : word := W#16#0;
    D_44 : word := W#16#1;
    D_45 : word := W#16#0;
    D_46 : word := W#16#0;
    D_47 : word := W#16#0;
    D_48 : word := W#16#0;
    D_49 : word := W#16#0;
    D_50 : word := W#16#0;
    D_51 : word := W#16#0;
    D_52 : word := W#16#0;
    D_53 : word := W#16#0;
    D_54 : word := W#16#0;
    D_55 : word := W#16#8000;
    D_56 : word := W#16#0;
    D_57 : word := W#16#0;
    D_58 : word := W#16#0;
    D_59 : word := W#16#4;
    D_60 : word := W#16#FE58;
    D_61 : word := W#16#0;
    D_62 : word := W#16#5;
    D_63 : word := W#16#4;
    D_64 : word := W#16#1;
    D_65 : word := W#16#0;
    D_66 : word := W#16#0;
    D_67 : word := W#16#0;
    D_68 : word := W#16#0;
    D_69 : word := W#16#0;
    D_70 : word := W#16#FE58;
    D_71 : word := W#16#0;
    D_72 : word := W#16#0;
    D_73 : word := W#16#0;
    D_74 : word := W#16#0;
    D_75 : word := W#16#0;
    D_76 : word := W#16#0;
    D_77 : word := W#16#0;
    D_78 : word := W#16#0;
    D_79 : word := W#16#0;
    D_80 : word := W#16#0;
    D_81 : word := W#16#0;
    D_82 : word := W#16#0;
    D_83 : word := W#16#0;
    D_84 : word := W#16#0;
    D_85 : word := W#16#0;
    D_86 : word := W#16#0;
    D_87 : word := W#16#0;
    D_88 : word := W#16#0;
    D_89 : word := W#16#0;
    D_90 : word := W#16#0;
    D_91 : word := W#16#0;
    D_92 : word := W#16#0;
    D_93 : word := W#16#0;
    D_94 : word := W#16#0;
    D_95 : word := W#16#0;
    D_96 : word := W#16#0;
    D_97 : word := W#16#0;
    D_98 : word := W#16#0;
    D_99 : word := W#16#0;
    D_100 : word := W#16#0;
    D_101 : word := W#16#0;
    D_102 : word := W#16#0;
    D_103 : word := W#16#0;
    D_104 : word := W#16#0;
    D_105 : word := W#16#0;
    D_106 : word := W#16#0;
    D_107 : word := W#16#0;
    D_108 : word := W#16#0;
    D_109 : word := W#16#0;
    D_110 : word := W#16#0;
    D_111 : word := W#16#0;
    D_112 : word := W#16#0;
    D_113 : word := W#16#0;
    D_114 : word := W#16#0;
    D_115 : word := W#16#0;
    D_116 : word := W#16#0;
    D_117 : word := W#16#0;
    D_118 : word := W#16#0;
    D_119 : word := W#16#0;
    D_120 : word := W#16#0;
  END_STRUCT
BEGIN

END_DATA_BLOCK

DATA_BLOCK DB 150


STRUCT
    D_0 : word := W#16#FC64;
    D_1 : word := W#16#0;
    D_2 : word := W#16#2B0;
    D_3 : word := W#16#5000;
    D_4 : word := W#16#36A;
    D_5 : word := W#16#4000;
    D_6 : word := W#16#758;
    D_7 : word := W#16#2200;
    D_8 : word := W#16#46C;
    D_9 : word := W#16#9800;
    D_10 : word := W#16#74C;
    D_11 : word := W#16#1300;
    D_12 : word := W#16#8000;
    D_13 : word := W#16#0;
    D_14 : word := W#16#44C;
    D_15 : word := W#16#A000;
    D_16 : word := W#16#58A;
    D_17 : word := W#16#D000;
    D_18 : word := W#16#768;
    D_19 : word := W#16#C900;
    D_20 : word := W#16#649;
    D_21 : word := W#16#3E00;
    D_22 : word := W#16#8000;
    D_23 : word := W#16#0;
    D_24 : word := W#16#37D;
    D_25 : word := W#16#0;
    D_26 : word := W#16#1B1;
    D_27 : word := W#16#E000;
    D_28 : word := W#16#1B1;
    D_29 : word := W#16#E000;
    D_30 : word := W#16#36D;
    D_31 : word := W#16#6000;
    D_32 : word := W#16#376;
    D_33 : word := W#16#2000;
    D_34 : word := W#16#490;
    D_35 : word := W#16#7000;
    D_36 : word := W#16#FE9C;
    D_37 : word := W#16#0;
    D_38 : word := W#16#FEB9;
    D_39 : word := W#16#E000;
    D_40 : word := W#16#FBB9;
    D_41 : word := W#16#0;
    D_42 : word := W#16#654;
    D_43 : word := W#16#0;
    D_44 : word := W#16#845;
    D_45 : word := W#16#2000;
    D_46 : word := W#16#449;
    D_47 : word := W#16#D000;
    D_48 : word := W#16#FF7F;
    D_49 : word := W#16#8000;
    D_50 : word := W#16#146;
    D_51 : word := W#16#5000;
    D_52 : word := W#16#FE57;
    D_53 : word := W#16#8000;
    D_54 : word := W#16#86;
    D_55 : word := W#16#2000;
    D_56 : word := W#16#FB9C;
    D_57 : word := W#16#0;
    D_58 : word := W#16#98;
    D_59 : word := W#16#E000;
    D_60 : word := W#16#1AB;
    D_61 : word := W#16#A000;
    D_62 : word := W#16#FB78;
    D_63 : word := W#16#0;
    D_64 : word := W#16#FE54;
    D_65 : word := W#16#4000;
    D_66 : word := W#16#FBB0;
    D_67 : word := W#16#0;
    D_68 : word := W#16#44F;
    D_69 : word := W#16#8400;
    D_70 : word := W#16#240;
    D_71 : word := W#16#0;
    D_72 : word := W#16#446;
    D_73 : word := W#16#7E00;
    D_74 : word := W#16#FC64;
    D_75 : word := W#16#0;
    D_76 : word := W#16#FC64;
    D_77 : word := W#16#0;
    D_78 : word := W#16#8000;
    D_79 : word := W#16#0;
    D_80 : word := W#16#35B;
    D_81 : word := W#16#6800;
    D_82 : word := W#16#FD64;
    D_83 : word := W#16#0;
    D_84 : word := W#16#15D;
    D_85 : word := W#16#C000;
    D_86 : word := W#16#398;
    D_87 : word := W#16#D500;
    D_88 : word := W#16#647;
    D_89 : word := W#16#2800;
    D_90 : word := W#16#545;
    D_91 : word := W#16#8800;
    D_92 : word := W#16#FC64;
    D_93 : word := W#16#0;
    D_94 : word := W#16#FE7D;
    D_95 : word := W#16#0;
    D_96 : word := W#16#240;
    D_97 : word := W#16#2800;
    D_98 : word := W#16#445;
    D_99 : word := W#16#200;
    D_100 : word := W#16#3BD;
    D_101 : word := W#16#CC00;
    D_102 : word := W#16#B51;
    D_103 : word := W#16#9C00;
    D_104 : word := W#16#8000;
    D_105 : word := W#16#0;
    D_106 : word := W#16#76A;
    D_107 : word := W#16#0;
    D_108 : word := W#16#76C;
    D_109 : word := W#16#0;
    D_110 : word := W#16#76E;
    D_111 : word := W#16#0;
    D_112 : word := W#16#749;
    D_113 : word := W#16#6300;
    D_114 : word := W#16#557;
    D_115 : word := W#16#E400;
    D_116 : word := W#16#55D;
    D_117 : word := W#16#C000;
    D_118 : word := W#16#54E;
    D_119 : word := W#16#E800;
    D_120 : word := W#16#8000;
    D_121 : word := W#16#0;
    D_122 : word := W#16#7D;
    D_123 : word := W#16#0;
    D_124 : word := W#16#376;
    D_125 : word := W#16#2C00;
    D_126 : word := W#16#451;
    D_127 : word := W#16#1E00;
    D_128 : word := W#16#479;
    D_129 : word := W#16#1800;
    D_130 : word := W#16#11E0;
    D_131 : word := W#16#0;
    D_132 : word := W#16#845;
    D_133 : word := W#16#3D00;
    D_134 : word := W#16#649;
    D_135 : word := W#16#3E00;
    D_136 : word := W#16#44B;
    D_137 : word := W#16#3800;
    D_138 : word := W#16#440;
    D_139 : word := W#16#CA00;
    D_140 : word := W#16#450;
    D_141 : word := W#16#5100;
    D_142 : word := W#16#240;
    D_143 : word := W#16#1400;
    D_144 : word := W#16#247;
    D_145 : word := W#16#D000;
    D_146 : word := W#16#259;
    D_147 : word := W#16#F00;
    D_148 : word := W#16#8000;
    D_149 : word := W#16#0;
    D_150 : word := W#16#8000;
    D_151 : word := W#16#0;
    D_152 : word := W#16#0;
    D_153 : word := W#16#0;
    D_154 : word := W#16#8000;
    D_155 : word := W#16#0;
    D_156 : word := W#16#8000;
    D_157 : word := W#16#0;
    D_158 : word := W#16#875;
    D_159 : word := W#16#8CCD;
    D_160 : word := W#16#443;
    D_161 : word := W#16#A300;
    D_162 : word := W#16#374;
    D_163 : word := W#16#9000;
    D_164 : word := W#16#448;
    D_165 : word := W#16#3D00;
    D_166 : word := W#16#78;
    D_167 : word := W#16#5900;
    D_168 : word := W#16#67;
    D_169 : word := W#16#A900;
    D_170 : word := W#16#140;
    D_171 : word := W#16#4000;
    D_172 : word := W#16#44B;
    D_173 : word := W#16#2800;
    D_174 : word := W#16#440;
    D_175 : word := W#16#C200;
    D_176 : word := W#16#450;
    D_177 : word := W#16#4400;
    D_178 : word := W#16#8000;
    D_179 : word := W#16#0;
    D_180 : word := W#16#B4D;
    D_181 : word := W#16#6100;
    D_182 : word := W#16#741;
    D_183 : word := W#16#4900;
    D_184 : word := W#16#B51;
    D_185 : word := W#16#7500;
    D_186 : word := W#16#8000;
    D_187 : word := W#16#0;
    D_188 : word := W#16#8000;
    D_189 : word := W#16#0;
    D_190 : word := W#16#8000;
    D_191 : word := W#16#0;
    D_192 : word := W#16#8000;
    D_193 : word := W#16#0;
    D_194 : word := W#16#8000;
    D_195 : word := W#16#0;
    D_196 : word := W#16#8000;
    D_197 : word := W#16#0;
    D_198 : word := W#16#8000;
    D_199 : word := W#16#0;
    D_200 : word := W#16#8000;
    D_201 : word := W#16#0;
    D_202 : word := W#16#8000;
    D_203 : word := W#16#0;
    D_204 : word := W#16#8000;
    D_205 : word := W#16#0;
    D_206 : word := W#16#8000;
    D_207 : word := W#16#0;
    D_208 : word := W#16#8000;
    D_209 : word := W#16#0;
    D_210 : word := W#16#8000;
    D_211 : word := W#16#0;
    D_212 : word := W#16#8000;
    D_213 : word := W#16#0;
    D_214 : word := W#16#8000;
    D_215 : word := W#16#0;
    D_216 : word := W#16#369;
    D_217 : word := W#16#999A;
    D_218 : word := W#16#369;
    D_219 : word := W#16#999A;
    D_220 : word := W#16#369;
    D_221 : word := W#16#999A;
    D_222 : word := W#16#260;
    D_223 : word := W#16#0;
    D_224 : word := W#16#260;
    D_225 : word := W#16#0;
    D_226 : word := W#16#260;
    D_227 : word := W#16#0;
    D_228 : word := W#16#8000;
    D_229 : word := W#16#0;
    D_230 : word := W#16#8000;
    D_231 : word := W#16#0;
  END_STRUCT
BEGIN

END_DATA_BLOCK

DATA_BLOCK DB 151


STRUCT
    D_0 : word := W#16#25D;
    D_1 : word := W#16#C000;
    D_2 : word := W#16#8000;
    D_3 : word := W#16#0;
    D_4 : word := W#16#744;
    D_5 : word := W#16#9300;
    D_6 : word := W#16#FF69;
    D_7 : word := W#16#8000;
    D_8 : word := W#16#847;
    D_9 : word := W#16#7C00;
    D_10 : word := W#16#B72;
    D_11 : word := W#16#0;
    D_12 : word := W#16#4B;
    D_13 : word := W#16#0;
    D_14 : word := W#16#2B0;
    D_15 : word := W#16#2800;
    D_16 : word := W#16#488;
    D_17 : word := W#16#1400;
    D_18 : word := W#16#676;
    D_19 : word := W#16#5C00;
    D_20 : word := W#16#8000;
    D_21 : word := W#16#0;
    D_22 : word := W#16#488;
    D_23 : word := W#16#3C00;
    D_24 : word := W#16#8000;
    D_25 : word := W#16#0;
    D_26 : word := W#16#8000;
    D_27 : word := W#16#0;
    D_28 : word := W#16#8000;
    D_29 : word := W#16#0;
    D_30 : word := W#16#8000;
    D_31 : word := W#16#0;
    D_32 : word := W#16#8000;
    D_33 : word := W#16#0;
    D_34 : word := W#16#8000;
    D_35 : word := W#16#0;
    D_36 : word := W#16#8000;
    D_37 : word := W#16#0;
    D_38 : word := W#16#8000;
    D_39 : word := W#16#0;
    D_40 : word := W#16#39F;
    D_41 : word := W#16#2000;
    D_42 : word := W#16#548;
    D_43 : word := W#16#A800;
    D_44 : word := W#16#FDBC;
    D_45 : word := W#16#3200;
    D_46 : word := W#16#83;
    D_47 : word := W#16#0;
    D_48 : word := W#16#65C;
    D_49 : word := W#16#F800;
    D_50 : word := W#16#9BD;
    D_51 : word := W#16#E300;
    D_52 : word := W#16#649;
    D_53 : word := W#16#4000;
    D_54 : word := W#16#475;
    D_55 : word := W#16#6000;
    D_56 : word := W#16#8000;
    D_57 : word := W#16#0;
    D_58 : word := W#16#8000;
    D_59 : word := W#16#0;
    D_60 : word := W#16#8000;
    D_61 : word := W#16#0;
    D_62 : word := W#16#8000;
    D_63 : word := W#16#0;
    D_64 : word := W#16#756;
    D_65 : word := W#16#6D00;
    D_66 : word := W#16#683;
    D_67 : word := W#16#3E00;
    D_68 : word := W#16#8000;
    D_69 : word := W#16#0;
    D_70 : word := W#16#8000;
    D_71 : word := W#16#0;
    D_72 : word := W#16#8000;
    D_73 : word := W#16#0;
    D_74 : word := W#16#8000;
    D_75 : word := W#16#0;
    D_76 : word := W#16#8000;
    D_77 : word := W#16#0;
    D_78 : word := W#16#8000;
    D_79 : word := W#16#0;
    D_80 : word := W#16#678;
    D_81 : word := W#16#E600;
    D_82 : word := W#16#94B;
    D_83 : word := W#16#4B00;
    D_84 : word := W#16#54B;
    D_85 : word := W#16#9600;
    D_86 : word := W#16#77D;
    D_87 : word := W#16#3200;
    D_88 : word := W#16#AA2;
    D_89 : word := W#16#6E00;
    D_90 : word := W#16#59C;
    D_91 : word := W#16#3200;
    D_92 : word := W#16#88F;
    D_93 : word := W#16#8C00;
    D_94 : word := W#16#25F;
    D_95 : word := W#16#5000;
    D_96 : word := W#16#7B4;
    D_97 : word := W#16#DA00;
    D_98 : word := W#16#355;
    D_99 : word := W#16#C000;
    D_100 : word := W#16#7B5;
    D_101 : word := W#16#6400;
    D_102 : word := W#16#59C;
    D_103 : word := W#16#0;
    D_104 : word := W#16#77E;
    D_105 : word := W#16#5700;
    D_106 : word := W#16#2AF;
    D_107 : word := W#16#D800;
    D_108 : word := W#16#2AF;
    D_109 : word := W#16#D800;
    D_110 : word := W#16#4B9;
    D_111 : word := W#16#DD00;
    D_112 : word := W#16#B5F;
    D_113 : word := W#16#7800;
    D_114 : word := W#16#8000;
    D_115 : word := W#16#0;
    D_116 : word := W#16#8000;
    D_117 : word := W#16#0;
    D_118 : word := W#16#8000;
    D_119 : word := W#16#0;
    D_120 : word := W#16#8000;
    D_121 : word := W#16#0;
    D_122 : word := W#16#8000;
    D_123 : word := W#16#0;
    D_124 : word := W#16#488;
    D_125 : word := W#16#1400;
    D_126 : word := W#16#59C;
    D_127 : word := W#16#0;
    D_128 : word := W#16#8000;
    D_129 : word := W#16#0;
    D_130 : word := W#16#0;
    D_131 : word := W#16#0;
    D_132 : word := W#16#8000;
    D_133 : word := W#16#0;
    D_134 : word := W#16#8000;
    D_135 : word := W#16#0;
    D_136 : word := W#16#8000;
    D_137 : word := W#16#0;
    D_138 : word := W#16#8000;
    D_139 : word := W#16#0;
    D_140 : word := W#16#8000;
    D_141 : word := W#16#0;
    D_142 : word := W#16#8000;
    D_143 : word := W#16#0;
  END_STRUCT
BEGIN

END_DATA_BLOCK

DATA_BLOCK DB 152


STRUCT
    D_0 : word := W#16#443;
    D_1 : word := W#16#8A00;
    D_2 : word := W#16#473;
    D_3 : word := W#16#C800;
    D_4 : word := W#16#797;
    D_5 : word := W#16#AD00;
    D_6 : word := W#16#55E;
    D_7 : word := W#16#1200;
    D_8 : word := W#16#764;
    D_9 : word := W#16#B400;
    D_10 : word := W#16#840;
    D_11 : word := W#16#3800;
    D_12 : word := W#16#842;
    D_13 : word := W#16#800;
    D_14 : word := W#16#46E;
    D_15 : word := W#16#F500;
    D_16 : word := W#16#857;
    D_17 : word := W#16#2300;
    D_18 : word := W#16#6B8;
    D_19 : word := W#16#D700;
    D_20 : word := W#16#765;
    D_21 : word := W#16#E900;
    D_22 : word := W#16#85B;
    D_23 : word := W#16#F600;
    D_24 : word := W#16#55E;
    D_25 : word := W#16#1200;
    D_26 : word := W#16#953;
    D_27 : word := W#16#3700;
    D_28 : word := W#16#95F;
    D_29 : word := W#16#2000;
    D_30 : word := W#16#956;
    D_31 : word := W#16#8800;
    D_32 : word := W#16#443;
    D_33 : word := W#16#8A00;
    D_34 : word := W#16#443;
    D_35 : word := W#16#8A00;
    D_36 : word := W#16#465;
    D_37 : word := W#16#4F00;
    D_38 : word := W#16#CB3;
    D_39 : word := W#16#8C00;
    D_40 : word := W#16#650;
    D_41 : word := W#16#6666;
    D_42 : word := W#16#CB3;
    D_43 : word := W#16#9000;
    D_44 : word := W#16#9B6;
    D_45 : word := W#16#E200;
    D_46 : word := W#16#CB7;
    D_47 : word := W#16#800;
    D_48 : word := W#16#567;
    D_49 : word := W#16#B800;
    D_50 : word := W#16#543;
    D_51 : word := W#16#8A00;
    D_52 : word := W#16#668;
    D_53 : word := W#16#6666;
    D_54 : word := W#16#36A;
    D_55 : word := W#16#2200;
    D_56 : word := W#16#956;
    D_57 : word := W#16#AF00;
    D_58 : word := W#16#75B;
    D_59 : word := W#16#A900;
    D_60 : word := W#16#356;
    D_61 : word := W#16#D600;
    D_62 : word := W#16#560;
    D_63 : word := W#16#7C00;
    D_64 : word := W#16#54F;
    D_65 : word := W#16#9900;
    D_66 : word := W#16#552;
    D_67 : word := W#16#300;
    D_68 : word := W#16#659;
    D_69 : word := W#16#3F00;
    D_70 : word := W#16#56A;
    D_71 : word := W#16#2200;
    D_72 : word := W#16#9A5;
    D_73 : word := W#16#D800;
    D_74 : word := W#16#649;
    D_75 : word := W#16#9100;
    D_76 : word := W#16#AAC;
    D_77 : word := W#16#7B00;
    D_78 : word := W#16#743;
    D_79 : word := W#16#8A00;
    D_80 : word := W#16#750;
    D_81 : word := W#16#3333;
    D_82 : word := W#16#752;
    D_83 : word := W#16#3333;
    D_84 : word := W#16#754;
    D_85 : word := W#16#3333;
    D_86 : word := W#16#756;
    D_87 : word := W#16#3333;
    D_88 : word := W#16#758;
    D_89 : word := W#16#3333;
    D_90 : word := W#16#75A;
    D_91 : word := W#16#3333;
    D_92 : word := W#16#75C;
    D_93 : word := W#16#3333;
    D_94 : word := W#16#75E;
    D_95 : word := W#16#3333;
    D_96 : word := W#16#760;
    D_97 : word := W#16#3333;
    D_98 : word := W#16#762;
    D_99 : word := W#16#3333;
    D_100 : word := W#16#450;
    D_101 : word := W#16#28F6;
    D_102 : word := W#16#451;
    D_103 : word := W#16#C28F;
    D_104 : word := W#16#453;
    D_105 : word := W#16#5C29;
    D_106 : word := W#16#454;
    D_107 : word := W#16#F5C3;
    D_108 : word := W#16#456;
    D_109 : word := W#16#8F5C;
    D_110 : word := W#16#458;
    D_111 : word := W#16#28F6;
    D_112 : word := W#16#459;
    D_113 : word := W#16#C28F;
    D_114 : word := W#16#45B;
    D_115 : word := W#16#5C29;
    D_116 : word := W#16#45C;
    D_117 : word := W#16#F5C3;
    D_118 : word := W#16#45E;
    D_119 : word := W#16#8F5C;
    D_120 : word := W#16#778;
    D_121 : word := W#16#3333;
    D_122 : word := W#16#77A;
    D_123 : word := W#16#3333;
    D_124 : word := W#16#77C;
    D_125 : word := W#16#3333;
    D_126 : word := W#16#77E;
    D_127 : word := W#16#3333;
    D_128 : word := W#16#840;
    D_129 : word := W#16#199A;
    D_130 : word := W#16#38A0;
    D_131 : word := W#16#0;
  END_STRUCT
BEGIN

END_DATA_BLOCK

DATA_BLOCK DB 179


STRUCT
    D_0 : word := W#16#67C;
    D_1 : word := W#16#8DD5;
    D_2 : word := W#16#544;
    D_3 : word := W#16#634C;
    D_4 : word := W#16#F962;
    D_5 : word := W#16#2EFF;
    D_6 : word := W#16#8000;
    D_7 : word := W#16#0;
    D_8 : word := W#16#8000;
    D_9 : word := W#16#0;
    D_10 : word := W#16#8000;
    D_11 : word := W#16#0;
    D_12 : word := W#16#8000;
    D_13 : word := W#16#0;
    D_14 : word := W#16#8000;
    D_15 : word := W#16#0;
    D_16 : word := W#16#8000;
    D_17 : word := W#16#0;
    D_18 : word := W#16#8000;
    D_19 : word := W#16#0;
    D_20 : word := W#16#8000;
    D_21 : word := W#16#0;
    D_22 : word := W#16#8000;
    D_23 : word := W#16#0;
    D_24 : word := W#16#8000;
    D_25 : word := W#16#0;
    D_26 : word := W#16#8000;
    D_27 : word := W#16#0;
    D_28 : word := W#16#8000;
    D_29 : word := W#16#0;
    D_30 : word := W#16#8000;
    D_31 : word := W#16#0;
    D_32 : word := W#16#8000;
    D_33 : word := W#16#0;
    D_34 : word := W#16#8000;
    D_35 : word := W#16#0;
    D_36 : word := W#16#8000;
    D_37 : word := W#16#0;
    D_38 : word := W#16#8000;
    D_39 : word := W#16#0;
    D_40 : word := W#16#8000;
    D_41 : word := W#16#0;
    D_42 : word := W#16#8000;
    D_43 : word := W#16#0;
    D_44 : word := W#16#8000;
    D_45 : word := W#16#0;
    D_46 : word := W#16#8000;
    D_47 : word := W#16#0;
    D_48 : word := W#16#8000;
    D_49 : word := W#16#0;
    D_50 : word := W#16#8000;
    D_51 : word := W#16#0;
  END_STRUCT
BEGIN

END_DATA_BLOCK

DATA_BLOCK DB 180


STRUCT
    D_0 : word := W#16#64;
    D_1 : word := W#16#FB7A;
    D_2 : word := W#16#E147;
    D_3 : word := W#16#664;
    D_4 : word := W#16#0;
    D_5 : word := W#16#468;
    D_6 : word := W#16#147A;
    D_7 : word := W#16#B46;
    D_8 : word := W#16#A000;
    D_9 : word := W#16#764;
    D_10 : word := W#16#0;
    D_11 : word := W#16#64;
    D_12 : word := W#16#0;
    D_13 : word := W#16#FF66;
    D_14 : word := W#16#6666;
    D_15 : word := W#16#360;
    D_16 : word := W#16#0;
    D_17 : word := W#16#FA51;
    D_18 : word := W#16#EB85;
    D_19 : word := W#16#C7D;
    D_20 : word := W#16#0;
    D_21 : word := W#16#8000;
    D_22 : word := W#16#0;
    D_23 : word := W#16#0;
    D_24 : word := W#16#0;
    D_25 : word := W#16#FFAE;
    D_26 : word := W#16#147B;
    D_27 : word := W#16#44D;
    D_28 : word := W#16#3333;
    D_29 : word := W#16#FB51;
    D_30 : word := W#16#EB85;
    D_31 : word := W#16#180;
    D_32 : word := W#16#6;
    D_33 : word := W#16#764;
    D_34 : word := W#16#0;
    D_35 : word := W#16#0;
    D_36 : word := W#16#1;
    D_37 : word := W#16#140;
    D_38 : word := W#16#0;
    D_39 : word := W#16#450;
    D_40 : word := W#16#0;
    D_41 : word := W#16#FA51;
    D_42 : word := W#16#EB85;
    D_43 : word := W#16#A42;
    D_44 : word := W#16#4000;
    D_45 : word := W#16#44F;
    D_46 : word := W#16#FF00;
    D_47 : word := W#16#A;
    D_48 : word := W#16#0;
    D_49 : word := W#16#8000;
    D_50 : word := W#16#0;
    D_51 : word := W#16#8000;
    D_52 : word := W#16#0;
    D_53 : word := W#16#8000;
    D_54 : word := W#16#0;
    D_55 : word := W#16#8000;
    D_56 : word := W#16#0;
    D_57 : word := W#16#8000;
    D_58 : word := W#16#0;
    D_59 : word := W#16#0;
    D_60 : word := W#16#0;
    D_61 : word := W#16#FE94;
    D_62 : word := W#16#7AE2;
    D_63 : word := W#16#470;
    D_64 : word := W#16#0;
    D_65 : word := W#16#340;
    D_66 : word := W#16#28F5;
    D_67 : word := W#16#65A;
    D_68 : word := W#16#0;
    D_69 : word := W#16#764;
    D_70 : word := W#16#0;
    D_71 : word := W#16#0;
    D_72 : word := W#16#1;
    D_73 : word := W#16#B9;
    D_74 : word := W#16#999A;
    D_75 : word := W#16#640;
    D_76 : word := W#16#0;
    D_77 : word := W#16#450;
    D_78 : word := W#16#147A;
    D_79 : word := W#16#664;
    D_80 : word := W#16#0;
    D_81 : word := W#16#64F;
    D_82 : word := W#16#FF00;
    D_83 : word := W#16#28;
    D_84 : word := W#16#0;
    D_85 : word := W#16#3AC;
    D_86 : word := W#16#0;
    D_87 : word := W#16#640;
    D_88 : word := W#16#0;
    D_89 : word := W#16#368;
    D_90 : word := W#16#0;
    D_91 : word := W#16#668;
    D_92 : word := W#16#0;
    D_93 : word := W#16#64F;
    D_94 : word := W#16#FF00;
    D_95 : word := W#16#28;
    D_96 : word := W#16#0;
    D_97 : word := W#16#FE94;
    D_98 : word := W#16#7AE2;
    D_99 : word := W#16#470;
    D_100 : word := W#16#0;
    D_101 : word := W#16#E085;
    D_102 : word := W#16#1EB9;
    D_103 : word := W#16#FD66;
    D_104 : word := W#16#659B;
    D_105 : word := W#16#764;
    D_106 : word := W#16#0;
    D_107 : word := W#16#64;
    D_108 : word := W#16#0;
    D_109 : word := W#16#FD66;
    D_110 : word := W#16#6666;
    D_111 : word := W#16#470;
    D_112 : word := W#16#0;
    D_113 : word := W#16#FA51;
    D_114 : word := W#16#EB8A;
    D_115 : word := W#16#F4E;
    D_116 : word := W#16#200;
    D_117 : word := W#16#764;
    D_118 : word := W#16#0;
    D_119 : word := W#16#46;
    D_120 : word := W#16#1;
    D_121 : word := W#16#FD66;
    D_122 : word := W#16#6666;
    D_123 : word := W#16#470;
    D_124 : word := W#16#0;
    D_125 : word := W#16#FA51;
    D_126 : word := W#16#EB85;
    D_127 : word := W#16#E75;
    D_128 : word := W#16#3000;
    D_129 : word := W#16#764;
    D_130 : word := W#16#0;
    D_131 : word := W#16#64;
    D_132 : word := W#16#1;
    D_133 : word := W#16#FD99;
    D_134 : word := W#16#999A;
    D_135 : word := W#16#44D;
    D_136 : word := W#16#3333;
    D_137 : word := W#16#FB51;
    D_138 : word := W#16#EB85;
    D_139 : word := W#16#EC99;
    D_140 : word := W#16#9AF5;
    D_141 : word := W#16#64F;
    D_142 : word := W#16#FF00;
    D_143 : word := W#16#28;
    D_144 : word := W#16#0;
    D_145 : word := W#16#376;
    D_146 : word := W#16#0;
    D_147 : word := W#16#65A;
    D_148 : word := W#16#0;
    D_149 : word := W#16#45A;
    D_150 : word := W#16#0;
    D_151 : word := W#16#378;
    D_152 : word := W#16#0;
    D_153 : word := W#16#8000;
    D_154 : word := W#16#0;
    D_155 : word := W#16#0;
    D_156 : word := W#16#0;
    D_157 : word := W#16#376;
    D_158 : word := W#16#0;
    D_159 : word := W#16#65A;
    D_160 : word := W#16#0;
    D_161 : word := W#16#45A;
    D_162 : word := W#16#0;
    D_163 : word := W#16#370;
    D_164 : word := W#16#0;
    D_165 : word := W#16#8000;
    D_166 : word := W#16#0;
    D_167 : word := W#16#0;
    D_168 : word := W#16#0;
    D_169 : word := W#16#376;
    D_170 : word := W#16#0;
    D_171 : word := W#16#65A;
    D_172 : word := W#16#0;
    D_173 : word := W#16#45A;
    D_174 : word := W#16#0;
    D_175 : word := W#16#36F;
    D_176 : word := W#16#FFFB;
    D_177 : word := W#16#8000;
    D_178 : word := W#16#0;
    D_179 : word := W#16#64;
    D_180 : word := W#16#1;
    D_181 : word := W#16#376;
    D_182 : word := W#16#0;
    D_183 : word := W#16#75E;
    D_184 : word := W#16#FFFF;
    D_185 : word := W#16#558;
    D_186 : word := W#16#0;
    D_187 : word := W#16#37C;
    D_188 : word := W#16#CCCA;
    D_189 : word := W#16#8000;
    D_190 : word := W#16#0;
    D_191 : word := W#16#0;
    D_192 : word := W#16#0;
    D_193 : word := W#16#376;
    D_194 : word := W#16#0;
    D_195 : word := W#16#75F;
    D_196 : word := W#16#0;
    D_197 : word := W#16#664;
    D_198 : word := W#16#0;
    D_199 : word := W#16#440;
    D_200 : word := W#16#0;
    D_201 : word := W#16#8000;
    D_202 : word := W#16#0;
    D_203 : word := W#16#0;
    D_204 : word := W#16#0;
    D_205 : word := W#16#3AD;
    D_206 : word := W#16#1EB9;
    D_207 : word := W#16#758;
    D_208 : word := W#16#0;
    D_209 : word := W#16#470;
    D_210 : word := W#16#0;
    D_211 : word := W#16#B4C;
    D_212 : word := W#16#7000;
    D_213 : word := W#16#8000;
    D_214 : word := W#16#0;
    D_215 : word := W#16#0;
    D_216 : word := W#16#0;
    D_217 : word := W#16#2B4;
    D_218 : word := W#16#E14A;
    D_219 : word := W#16#44F;
    D_220 : word := W#16#FFFC;
    D_221 : word := W#16#341;
    D_222 : word := W#16#C28F;
    D_223 : word := W#16#478;
    D_224 : word := W#16#0;
    D_225 : word := W#16#764;
    D_226 : word := W#16#0;
    D_227 : word := W#16#A;
    D_228 : word := W#16#0;
    D_229 : word := W#16#29C;
    D_230 : word := W#16#B733;
    D_231 : word := W#16#44F;
    D_232 : word := W#16#FFFE;
    D_233 : word := W#16#340;
    D_234 : word := W#16#28F5;
    D_235 : word := W#16#470;
    D_236 : word := W#16#0;
    D_237 : word := W#16#44F;
    D_238 : word := W#16#FF00;
    D_239 : word := W#16#A;
    D_240 : word := W#16#0;
    D_241 : word := W#16#4A8;
    D_242 : word := W#16#0;
    D_243 : word := W#16#75E;
    D_244 : word := W#16#0;
    D_245 : word := W#16#550;
    D_246 : word := W#16#A3D;
    D_247 : word := W#16#666;
    D_248 : word := W#16#0;
    D_249 : word := W#16#764;
    D_250 : word := W#16#0;
    D_251 : word := W#16#A;
    D_252 : word := W#16#1;
  END_STRUCT
BEGIN

END_DATA_BLOCK

DATA_BLOCK DB 181


STRUCT
    D_0 : word := W#16#0;
    D_1 : word := W#16#180;
    D_2 : word := W#16#0;
    D_3 : word := W#16#240;
    D_4 : word := W#16#0;
    D_5 : word := W#16#240;
    D_6 : word := W#16#F5C2;
    D_7 : word := W#16#647;
    D_8 : word := W#16#0;
    D_9 : word := W#16#8000;
    D_10 : word := W#16#0;
    D_11 : word := W#16#0;
    D_12 : word := W#16#0;
    D_13 : word := W#16#58B;
    D_14 : word := W#16#999B;
    D_15 : word := W#16#448;
    D_16 : word := W#16#0;
    D_17 : word := W#16#FB51;
    D_18 : word := W#16#EB85;
    D_19 : word := W#16#458;
    D_20 : word := W#16#0;
    D_21 : word := W#16#8000;
    D_22 : word := W#16#0;
    D_23 : word := W#16#0;
    D_24 : word := W#16#1;
    D_25 : word := W#16#4C;
    D_26 : word := W#16#CC99;
    D_27 : word := W#16#350;
    D_28 : word := W#16#0;
    D_29 : word := W#16#FA5A;
    D_30 : word := W#16#39F5;
    D_31 : word := W#16#4C;
    D_32 : word := W#16#CCC4;
    D_33 : word := W#16#579;
    D_34 : word := W#16#DB00;
    D_35 : word := W#16#0;
    D_36 : word := W#16#1;
    D_37 : word := W#16#FD51;
    D_38 : word := W#16#EB85;
    D_39 : word := W#16#240;
    D_40 : word := W#16#0;
    D_41 : word := W#16#240;
    D_42 : word := W#16#F5C2;
    D_43 : word := W#16#460;
    D_44 : word := W#16#0;
    D_45 : word := W#16#74F;
    D_46 : word := W#16#FF00;
    D_47 : word := W#16#50;
    D_48 : word := W#16#0;
    D_49 : word := W#16#8000;
    D_50 : word := W#16#0;
    D_51 : word := W#16#8000;
    D_52 : word := W#16#0;
    D_53 : word := W#16#8000;
    D_54 : word := W#16#0;
    D_55 : word := W#16#8000;
    D_56 : word := W#16#0;
    D_57 : word := W#16#8000;
    D_58 : word := W#16#0;
    D_59 : word := W#16#0;
    D_60 : word := W#16#0;
    D_61 : word := W#16#FB46;
    D_62 : word := W#16#FB85;
    D_63 : word := W#16#74F;
    D_64 : word := W#16#9998;
    D_65 : word := W#16#34F;
    D_66 : word := W#16#FFF6;
    D_67 : word := W#16#564;
    D_68 : word := W#16#0;
    D_69 : word := W#16#8000;
    D_70 : word := W#16#0;
    D_71 : word := W#16#0;
    D_72 : word := W#16#0;
    D_73 : word := W#16#350;
    D_74 : word := W#16#0;
    D_75 : word := W#16#351;
    D_76 : word := W#16#9999;
    D_77 : word := W#16#FD66;
    D_78 : word := W#16#6666;
    D_79 : word := W#16#846;
    D_80 : word := W#16#0;
    D_81 : word := W#16#764;
    D_82 : word := W#16#0;
    D_83 : word := W#16#0;
    D_84 : word := W#16#1;
    D_85 : word := W#16#8000;
    D_86 : word := W#16#0;
    D_87 : word := W#16#8000;
    D_88 : word := W#16#0;
    D_89 : word := W#16#8000;
    D_90 : word := W#16#0;
    D_91 : word := W#16#8000;
    D_92 : word := W#16#0;
    D_93 : word := W#16#8000;
    D_94 : word := W#16#0;
    D_95 : word := W#16#8000;
    D_96 : word := W#16#0;
    D_97 : word := W#16#8000;
    D_98 : word := W#16#0;
    D_99 : word := W#16#8000;
    D_100 : word := W#16#0;
    D_101 : word := W#16#658;
    D_102 : word := W#16#0;
    D_103 : word := W#16#875;
    D_104 : word := W#16#8000;
    D_105 : word := W#16#A63;
    D_106 : word := W#16#DFFF;
    D_107 : word := W#16#54F;
    D_108 : word := W#16#FFFF;
    D_109 : word := W#16#36E;
    D_110 : word := W#16#6664;
    D_111 : word := W#16#357;
    D_112 : word := W#16#FFFD;
    D_113 : word := W#16#2;
    D_114 : word := W#16#0;
    D_115 : word := W#16#751;
    D_116 : word := W#16#AF31;
    D_117 : word := W#16#751;
    D_118 : word := W#16#AF31;
    D_119 : word := W#16#FD66;
    D_120 : word := W#16#61CA;
    D_121 : word := W#16#658;
    D_122 : word := W#16#0;
    D_123 : word := W#16#8000;
    D_124 : word := W#16#0;
    D_125 : word := W#16#450;
    D_126 : word := W#16#0;
    D_127 : word := W#16#8000;
    D_128 : word := W#16#0;
    D_129 : word := W#16#8000;
    D_130 : word := W#16#0;
    D_131 : word := W#16#8000;
    D_132 : word := W#16#0;
    D_133 : word := W#16#8000;
    D_134 : word := W#16#0;
    D_135 : word := W#16#8000;
    D_136 : word := W#16#0;
    D_137 : word := W#16#8000;
    D_138 : word := W#16#0;
    D_139 : word := W#16#8000;
    D_140 : word := W#16#0;
    D_141 : word := W#16#8000;
    D_142 : word := W#16#0;
    D_143 : word := W#16#8000;
    D_144 : word := W#16#0;
    D_145 : word := W#16#8000;
    D_146 : word := W#16#0;
    D_147 : word := W#16#8000;
    D_148 : word := W#16#0;
    D_149 : word := W#16#8000;
    D_150 : word := W#16#0;
    D_151 : word := W#16#8000;
    D_152 : word := W#16#0;
    D_153 : word := W#16#8000;
    D_154 : word := W#16#0;
    D_155 : word := W#16#8000;
    D_156 : word := W#16#0;
    D_157 : word := W#16#8000;
    D_158 : word := W#16#0;
    D_159 : word := W#16#8000;
    D_160 : word := W#16#0;
    D_161 : word := W#16#8000;
    D_162 : word := W#16#0;
    D_163 : word := W#16#8000;
    D_164 : word := W#16#0;
    D_165 : word := W#16#8000;
    D_166 : word := W#16#0;
    D_167 : word := W#16#8000;
    D_168 : word := W#16#0;
    D_169 : word := W#16#8000;
    D_170 : word := W#16#0;
    D_171 : word := W#16#8000;
    D_172 : word := W#16#0;
    D_173 : word := W#16#8000;
    D_174 : word := W#16#0;
    D_175 : word := W#16#8000;
    D_176 : word := W#16#0;
    D_177 : word := W#16#8000;
    D_178 : word := W#16#0;
    D_179 : word := W#16#8000;
    D_180 : word := W#16#0;
    D_181 : word := W#16#8000;
    D_182 : word := W#16#0;
    D_183 : word := W#16#8000;
    D_184 : word := W#16#0;
    D_185 : word := W#16#8000;
    D_186 : word := W#16#0;
    D_187 : word := W#16#8000;
    D_188 : word := W#16#0;
    D_189 : word := W#16#8000;
    D_190 : word := W#16#0;
    D_191 : word := W#16#8000;
    D_192 : word := W#16#0;
    D_193 : word := W#16#8000;
    D_194 : word := W#16#0;
    D_195 : word := W#16#8000;
    D_196 : word := W#16#0;
    D_197 : word := W#16#8000;
    D_198 : word := W#16#0;
    D_199 : word := W#16#8000;
    D_200 : word := W#16#0;
    D_201 : word := W#16#8000;
    D_202 : word := W#16#0;
  END_STRUCT
BEGIN

END_DATA_BLOCK

DATA_BLOCK DB 182


STRUCT
    D_0 : word := W#16#0;
    D_1 : word := W#16#A4B;
    D_2 : word := W#16#0;
    D_3 : word := W#16#A44;
    D_4 : word := W#16#C000;
    D_5 : word := W#16#A44;
    D_6 : word := W#16#C000;
    D_7 : word := W#16#A44;
    D_8 : word := W#16#C000;
  END_STRUCT
BEGIN

END_DATA_BLOCK

DATA_BLOCK DB 200


STRUCT
    D_0 : word := W#16#0;
    D_1 : word := W#16#8000;
    D_2 : word := W#16#0;
    D_3 : word := W#16#8000;
    D_4 : word := W#16#0;
    D_5 : word := W#16#8000;
    D_6 : word := W#16#0;
    D_7 : word := W#16#8000;
    D_8 : word := W#16#0;
    D_9 : word := W#16#8000;
    D_10 : word := W#16#0;
    D_11 : word := W#16#0;
    D_12 : word := W#16#8000;
    D_13 : word := W#16#0;
    D_14 : word := W#16#8000;
    D_15 : word := W#16#0;
    D_16 : word := W#16#8000;
    D_17 : word := W#16#0;
    D_18 : word := W#16#0;
    D_19 : word := W#16#0;
    D_20 : word := W#16#0;
    D_21 : word := W#16#0;
    D_22 : word := W#16#8000;
    D_23 : word := W#16#0;
    D_24 : word := W#16#0;
    D_25 : word := W#16#8000;
    D_26 : word := W#16#0;
    D_27 : word := W#16#8000;
    D_28 : word := W#16#0;
    D_29 : word := W#16#0;
    D_30 : word := W#16#8000;
    D_31 : word := W#16#0;
    D_32 : word := W#16#8000;
    D_33 : word := W#16#0;
    D_34 : word := W#16#8000;
    D_35 : word := W#16#0;
    D_36 : word := W#16#8000;
    D_37 : word := W#16#0;
    D_38 : word := W#16#8000;
    D_39 : word := W#16#0;
    D_40 : word := W#16#8000;
    D_41 : word := W#16#0;
    D_42 : word := W#16#0;
    D_43 : word := W#16#F940;
    D_44 : word := W#16#0;
    D_45 : word := W#16#0;
    D_46 : word := W#16#8000;
    D_47 : word := W#16#0;
    D_48 : word := W#16#0;
  END_STRUCT
BEGIN

END_DATA_BLOCK

DATA_BLOCK DB 201


STRUCT
    D_0 : word := W#16#0;
    D_1 : word := W#16#FB7A;
    D_2 : word := W#16#E147;
    D_3 : word := W#16#140;
    D_4 : word := W#16#0;
    D_5 : word := W#16#FD41;
    D_6 : word := W#16#8800;
    D_7 : word := W#16#341;
    D_8 : word := W#16#C00;
    D_9 : word := W#16#45A;
    D_10 : word := W#16#6600;
    D_11 : word := W#16#1E0;
    D_12 : word := W#16#140;
    D_13 : word := W#16#0;
    D_14 : word := W#16#140;
    D_15 : word := W#16#0;
    D_16 : word := W#16#8000;
    D_17 : word := W#16#0;
    D_18 : word := W#16#0;
    D_19 : word := W#16#0;
    D_20 : word := W#16#300;
    D_21 : word := W#16#0;
    D_22 : word := W#16#175;
    D_23 : word := W#16#B400;
    D_24 : word := W#16#0;
    D_25 : word := W#16#0;
    D_26 : word := W#16#0;
    D_27 : word := W#16#0;
    D_28 : word := W#16#0;
    D_29 : word := W#16#0;
    D_30 : word := W#16#0;
    D_31 : word := W#16#0;
    D_32 : word := W#16#0;
    D_33 : word := W#16#0;
    D_34 : word := W#16#0;
    D_35 : word := W#16#0;
    D_36 : word := W#16#0;
    D_37 : word := W#16#0;
    D_38 : word := W#16#0;
    D_39 : word := W#16#0;
    D_40 : word := W#16#0;
    D_41 : word := W#16#0;
    D_42 : word := W#16#0;
    D_43 : word := W#16#0;
    D_44 : word := W#16#140;
    D_45 : word := W#16#0;
    D_46 : word := W#16#140;
    D_47 : word := W#16#0;
    D_48 : word := W#16#7FFF;
  END_STRUCT
BEGIN

END_DATA_BLOCK

DATA_BLOCK DB 202


STRUCT
    D_0 : word := W#16#0;
    D_1 : word := W#16#FF66;
    D_2 : word := W#16#6666;
    D_3 : word := W#16#140;
    D_4 : word := W#16#0;
    D_5 : word := W#16#FD55;
    D_6 : word := W#16#5400;
    D_7 : word := W#16#FB51;
    D_8 : word := W#16#EB00;
    D_9 : word := W#16#66;
    D_10 : word := W#16#6600;
    D_11 : word := W#16#1E0;
    D_12 : word := W#16#8000;
    D_13 : word := W#16#0;
    D_14 : word := W#16#140;
    D_15 : word := W#16#0;
    D_16 : word := W#16#8000;
    D_17 : word := W#16#0;
    D_18 : word := W#16#0;
    D_19 : word := W#16#0;
    D_20 : word := W#16#300;
    D_21 : word := W#16#0;
    D_22 : word := W#16#F863;
    D_23 : word := W#16#3300;
    D_24 : word := W#16#0;
    D_25 : word := W#16#0;
    D_26 : word := W#16#0;
    D_27 : word := W#16#0;
    D_28 : word := W#16#0;
    D_29 : word := W#16#0;
    D_30 : word := W#16#0;
    D_31 : word := W#16#0;
    D_32 : word := W#16#0;
    D_33 : word := W#16#0;
    D_34 : word := W#16#0;
    D_35 : word := W#16#0;
    D_36 : word := W#16#0;
    D_37 : word := W#16#0;
    D_38 : word := W#16#0;
    D_39 : word := W#16#0;
    D_40 : word := W#16#0;
    D_41 : word := W#16#0;
    D_42 : word := W#16#0;
    D_43 : word := W#16#0;
    D_44 : word := W#16#0;
    D_45 : word := W#16#0;
    D_46 : word := W#16#0;
    D_47 : word := W#16#0;
    D_48 : word := W#16#0;
  END_STRUCT
BEGIN

END_DATA_BLOCK

DATA_BLOCK DB 203


STRUCT
    D_0 : word := W#16#0;
    D_1 : word := W#16#FFAE;
    D_2 : word := W#16#147B;
    D_3 : word := W#16#140;
    D_4 : word := W#16#0;
    D_5 : word := W#16#FC6A;
    D_6 : word := W#16#1C00;
    D_7 : word := W#16#FC51;
    D_8 : word := W#16#EB00;
    D_9 : word := W#16#FE99;
    D_10 : word := W#16#9A00;
    D_11 : word := W#16#1E1;
    D_12 : word := W#16#8000;
    D_13 : word := W#16#0;
    D_14 : word := W#16#140;
    D_15 : word := W#16#0;
    D_16 : word := W#16#8000;
    D_17 : word := W#16#0;
    D_18 : word := W#16#0;
    D_19 : word := W#16#0;
    D_20 : word := W#16#1;
    D_21 : word := W#16#0;
    D_22 : word := W#16#F860;
    D_23 : word := W#16#0;
    D_24 : word := W#16#0;
    D_25 : word := W#16#0;
    D_26 : word := W#16#0;
    D_27 : word := W#16#0;
    D_28 : word := W#16#0;
    D_29 : word := W#16#0;
    D_30 : word := W#16#0;
    D_31 : word := W#16#0;
    D_32 : word := W#16#0;
    D_33 : word := W#16#0;
    D_34 : word := W#16#0;
    D_35 : word := W#16#0;
    D_36 : word := W#16#E194;
    D_37 : word := W#16#7C00;
    D_38 : word := W#16#FE98;
    D_39 : word := W#16#1A00;
    D_40 : word := W#16#8000;
    D_41 : word := W#16#0;
    D_42 : word := W#16#0;
    D_43 : word := W#16#0;
    D_44 : word := W#16#140;
    D_45 : word := W#16#4200;
    D_46 : word := W#16#140;
    D_47 : word := W#16#0;
    D_48 : word := W#16#7FFF;
  END_STRUCT
BEGIN

END_DATA_BLOCK

DATA_BLOCK DB 204


STRUCT
    D_0 : word := W#16#0;
    D_1 : word := W#16#140;
    D_2 : word := W#16#0;
    D_3 : word := W#16#140;
    D_4 : word := W#16#0;
    D_5 : word := W#16#FF51;
    D_6 : word := W#16#EB00;
    D_7 : word := W#16#F866;
    D_8 : word := W#16#6600;
    D_9 : word := W#16#FF71;
    D_10 : word := W#16#1000;
    D_11 : word := W#16#1E0;
    D_12 : word := W#16#FD66;
    D_13 : word := W#16#6600;
    D_14 : word := W#16#140;
    D_15 : word := W#16#0;
    D_16 : word := W#16#8000;
    D_17 : word := W#16#0;
    D_18 : word := W#16#0;
    D_19 : word := W#16#0;
    D_20 : word := W#16#300;
    D_21 : word := W#16#0;
    D_22 : word := W#16#FE4E;
    D_23 : word := W#16#7900;
    D_24 : word := W#16#0;
    D_25 : word := W#16#0;
    D_26 : word := W#16#0;
    D_27 : word := W#16#0;
    D_28 : word := W#16#0;
    D_29 : word := W#16#0;
    D_30 : word := W#16#0;
    D_31 : word := W#16#0;
    D_32 : word := W#16#0;
    D_33 : word := W#16#0;
    D_34 : word := W#16#0;
    D_35 : word := W#16#0;
    D_36 : word := W#16#0;
    D_37 : word := W#16#0;
    D_38 : word := W#16#0;
    D_39 : word := W#16#0;
    D_40 : word := W#16#0;
    D_41 : word := W#16#0;
    D_42 : word := W#16#0;
    D_43 : word := W#16#0;
    D_44 : word := W#16#FD66;
    D_45 : word := W#16#6600;
    D_46 : word := W#16#FD66;
    D_47 : word := W#16#6600;
    D_48 : word := W#16#CCC;
  END_STRUCT
BEGIN

END_DATA_BLOCK

DATA_BLOCK DB 205


STRUCT
    D_0 : word := W#16#0;
    D_1 : word := W#16#8000;
    D_2 : word := W#16#0;
    D_3 : word := W#16#8000;
    D_4 : word := W#16#0;
    D_5 : word := W#16#8000;
    D_6 : word := W#16#0;
    D_7 : word := W#16#8000;
    D_8 : word := W#16#0;
    D_9 : word := W#16#8000;
    D_10 : word := W#16#0;
    D_11 : word := W#16#0;
    D_12 : word := W#16#8000;
    D_13 : word := W#16#0;
    D_14 : word := W#16#8000;
    D_15 : word := W#16#0;
    D_16 : word := W#16#8000;
    D_17 : word := W#16#0;
    D_18 : word := W#16#0;
    D_19 : word := W#16#0;
    D_20 : word := W#16#0;
    D_21 : word := W#16#0;
    D_22 : word := W#16#0;
    D_23 : word := W#16#0;
    D_24 : word := W#16#0;
    D_25 : word := W#16#0;
    D_26 : word := W#16#0;
    D_27 : word := W#16#0;
    D_28 : word := W#16#0;
    D_29 : word := W#16#0;
    D_30 : word := W#16#0;
    D_31 : word := W#16#0;
    D_32 : word := W#16#0;
    D_33 : word := W#16#0;
    D_34 : word := W#16#0;
    D_35 : word := W#16#0;
    D_36 : word := W#16#0;
    D_37 : word := W#16#0;
    D_38 : word := W#16#0;
    D_39 : word := W#16#0;
    D_40 : word := W#16#0;
    D_41 : word := W#16#0;
    D_42 : word := W#16#0;
    D_43 : word := W#16#0;
    D_44 : word := W#16#0;
    D_45 : word := W#16#0;
    D_46 : word := W#16#0;
    D_47 : word := W#16#0;
    D_48 : word := W#16#0;
  END_STRUCT
BEGIN

END_DATA_BLOCK

DATA_BLOCK DB 206


STRUCT
    D_0 : word := W#16#0;
    D_1 : word := W#16#FE94;
    D_2 : word := W#16#7AE2;
    D_3 : word := W#16#140;
    D_4 : word := W#16#0;
    D_5 : word := W#16#FC75;
    D_6 : word := W#16#600;
    D_7 : word := W#16#350;
    D_8 : word := W#16#3200;
    D_9 : word := W#16#FF73;
    D_10 : word := W#16#3200;
    D_11 : word := W#16#1E1;
    D_12 : word := W#16#8000;
    D_13 : word := W#16#0;
    D_14 : word := W#16#140;
    D_15 : word := W#16#0;
    D_16 : word := W#16#8000;
    D_17 : word := W#16#0;
    D_18 : word := W#16#0;
    D_19 : word := W#16#0;
    D_20 : word := W#16#1;
    D_21 : word := W#16#0;
    D_22 : word := W#16#52;
    D_23 : word := W#16#E000;
    D_24 : word := W#16#0;
    D_25 : word := W#16#0;
    D_26 : word := W#16#0;
    D_27 : word := W#16#0;
    D_28 : word := W#16#0;
    D_29 : word := W#16#0;
    D_30 : word := W#16#0;
    D_31 : word := W#16#0;
    D_32 : word := W#16#0;
    D_33 : word := W#16#0;
    D_34 : word := W#16#0;
    D_35 : word := W#16#0;
    D_36 : word := W#16#7C;
    D_37 : word := W#16#B800;
    D_38 : word := W#16#FE9A;
    D_39 : word := W#16#E400;
    D_40 : word := W#16#FF42;
    D_41 : word := W#16#9C00;
    D_42 : word := W#16#0;
    D_43 : word := W#16#0;
    D_44 : word := W#16#14D;
    D_45 : word := W#16#BB00;
    D_46 : word := W#16#140;
    D_47 : word := W#16#0;
    D_48 : word := W#16#7FFF;
  END_STRUCT
BEGIN

END_DATA_BLOCK

DATA_BLOCK DB 207


STRUCT
    D_0 : word := W#16#0;
    D_1 : word := W#16#B9;
    D_2 : word := W#16#999A;
    D_3 : word := W#16#140;
    D_4 : word := W#16#0;
    D_5 : word := W#16#FB66;
    D_6 : word := W#16#6600;
    D_7 : word := W#16#464;
    D_8 : word := W#16#1800;
    D_9 : word := W#16#40;
    D_10 : word := W#16#0;
    D_11 : word := W#16#1E0;
    D_12 : word := W#16#FF66;
    D_13 : word := W#16#6600;
    D_14 : word := W#16#140;
    D_15 : word := W#16#0;
    D_16 : word := W#16#8000;
    D_17 : word := W#16#0;
    D_18 : word := W#16#0;
    D_19 : word := W#16#0;
    D_20 : word := W#16#300;
    D_21 : word := W#16#0;
    D_22 : word := W#16#FB9A;
    D_23 : word := W#16#0;
    D_24 : word := W#16#0;
    D_25 : word := W#16#0;
    D_26 : word := W#16#0;
    D_27 : word := W#16#0;
    D_28 : word := W#16#0;
    D_29 : word := W#16#0;
    D_30 : word := W#16#0;
    D_31 : word := W#16#0;
    D_32 : word := W#16#0;
    D_33 : word := W#16#0;
    D_34 : word := W#16#0;
    D_35 : word := W#16#0;
    D_36 : word := W#16#0;
    D_37 : word := W#16#0;
    D_38 : word := W#16#0;
    D_39 : word := W#16#0;
    D_40 : word := W#16#0;
    D_41 : word := W#16#0;
    D_42 : word := W#16#0;
    D_43 : word := W#16#0;
    D_44 : word := W#16#FF66;
    D_45 : word := W#16#6600;
    D_46 : word := W#16#FF66;
    D_47 : word := W#16#6600;
    D_48 : word := W#16#3333;
  END_STRUCT
BEGIN

END_DATA_BLOCK

DATA_BLOCK DB 208


STRUCT
    D_0 : word := W#16#0;
    D_1 : word := W#16#3AC;
    D_2 : word := W#16#0;
    D_3 : word := W#16#140;
    D_4 : word := W#16#0;
    D_5 : word := W#16#FB66;
    D_6 : word := W#16#6600;
    D_7 : word := W#16#441;
    D_8 : word := W#16#0;
    D_9 : word := W#16#42;
    D_10 : word := W#16#8F00;
    D_11 : word := W#16#1E0;
    D_12 : word := W#16#FF66;
    D_13 : word := W#16#6600;
    D_14 : word := W#16#140;
    D_15 : word := W#16#0;
    D_16 : word := W#16#8000;
    D_17 : word := W#16#0;
    D_18 : word := W#16#0;
    D_19 : word := W#16#0;
    D_20 : word := W#16#300;
    D_21 : word := W#16#0;
    D_22 : word := W#16#FD44;
    D_23 : word := W#16#0;
    D_24 : word := W#16#0;
    D_25 : word := W#16#0;
    D_26 : word := W#16#0;
    D_27 : word := W#16#0;
    D_28 : word := W#16#0;
    D_29 : word := W#16#0;
    D_30 : word := W#16#0;
    D_31 : word := W#16#0;
    D_32 : word := W#16#0;
    D_33 : word := W#16#0;
    D_34 : word := W#16#0;
    D_35 : word := W#16#0;
    D_36 : word := W#16#0;
    D_37 : word := W#16#0;
    D_38 : word := W#16#0;
    D_39 : word := W#16#0;
    D_40 : word := W#16#0;
    D_41 : word := W#16#0;
    D_42 : word := W#16#0;
    D_43 : word := W#16#0;
    D_44 : word := W#16#FF66;
    D_45 : word := W#16#6600;
    D_46 : word := W#16#FF66;
    D_47 : word := W#16#6600;
    D_48 : word := W#16#3333;
  END_STRUCT
BEGIN

END_DATA_BLOCK

DATA_BLOCK DB 209


STRUCT
    D_0 : word := W#16#0;
    D_1 : word := W#16#FE94;
    D_2 : word := W#16#7AE2;
    D_3 : word := W#16#140;
    D_4 : word := W#16#0;
    D_5 : word := W#16#FC49;
    D_6 : word := W#16#2400;
    D_7 : word := W#16#E185;
    D_8 : word := W#16#1E00;
    D_9 : word := W#16#F951;
    D_10 : word := W#16#EA00;
    D_11 : word := W#16#1E0;
    D_12 : word := W#16#140;
    D_13 : word := W#16#0;
    D_14 : word := W#16#140;
    D_15 : word := W#16#0;
    D_16 : word := W#16#8000;
    D_17 : word := W#16#0;
    D_18 : word := W#16#0;
    D_19 : word := W#16#0;
    D_20 : word := W#16#300;
    D_21 : word := W#16#0;
    D_22 : word := W#16#FB66;
    D_23 : word := W#16#0;
    D_24 : word := W#16#0;
    D_25 : word := W#16#0;
    D_26 : word := W#16#0;
    D_27 : word := W#16#0;
    D_28 : word := W#16#0;
    D_29 : word := W#16#0;
    D_30 : word := W#16#0;
    D_31 : word := W#16#0;
    D_32 : word := W#16#0;
    D_33 : word := W#16#0;
    D_34 : word := W#16#0;
    D_35 : word := W#16#0;
    D_36 : word := W#16#0;
    D_37 : word := W#16#0;
    D_38 : word := W#16#0;
    D_39 : word := W#16#0;
    D_40 : word := W#16#0;
    D_41 : word := W#16#0;
    D_42 : word := W#16#0;
    D_43 : word := W#16#0;
    D_44 : word := W#16#140;
    D_45 : word := W#16#0;
    D_46 : word := W#16#140;
    D_47 : word := W#16#0;
    D_48 : word := W#16#7FFF;
  END_STRUCT
BEGIN

END_DATA_BLOCK

DATA_BLOCK DB 210


STRUCT
    D_0 : word := W#16#0;
    D_1 : word := W#16#FD66;
    D_2 : word := W#16#6666;
    D_3 : word := W#16#140;
    D_4 : word := W#16#0;
    D_5 : word := W#16#FC49;
    D_6 : word := W#16#2400;
    D_7 : word := W#16#FB51;
    D_8 : word := W#16#EB00;
    D_9 : word := W#16#7F;
    D_10 : word := W#16#CE00;
    D_11 : word := W#16#1E1;
    D_12 : word := W#16#59;
    D_13 : word := W#16#9800;
    D_14 : word := W#16#140;
    D_15 : word := W#16#0;
    D_16 : word := W#16#8000;
    D_17 : word := W#16#0;
    D_18 : word := W#16#0;
    D_19 : word := W#16#0;
    D_20 : word := W#16#1;
    D_21 : word := W#16#0;
    D_22 : word := W#16#F778;
    D_23 : word := W#16#0;
    D_24 : word := W#16#0;
    D_25 : word := W#16#0;
    D_26 : word := W#16#0;
    D_27 : word := W#16#0;
    D_28 : word := W#16#0;
    D_29 : word := W#16#0;
    D_30 : word := W#16#0;
    D_31 : word := W#16#0;
    D_32 : word := W#16#0;
    D_33 : word := W#16#0;
    D_34 : word := W#16#0;
    D_35 : word := W#16#0;
    D_36 : word := W#16#80A0;
    D_37 : word := W#16#200;
    D_38 : word := W#16#7F;
    D_39 : word := W#16#9200;
    D_40 : word := W#16#8000;
    D_41 : word := W#16#0;
    D_42 : word := W#16#0;
    D_43 : word := W#16#0;
    D_44 : word := W#16#140;
    D_45 : word := W#16#1600;
    D_46 : word := W#16#140;
    D_47 : word := W#16#0;
    D_48 : word := W#16#7FFF;
  END_STRUCT
BEGIN

END_DATA_BLOCK

DATA_BLOCK DB 211


STRUCT
    D_0 : word := W#16#0;
    D_1 : word := W#16#FD66;
    D_2 : word := W#16#6666;
    D_3 : word := W#16#140;
    D_4 : word := W#16#0;
    D_5 : word := W#16#FC49;
    D_6 : word := W#16#2400;
    D_7 : word := W#16#FB51;
    D_8 : word := W#16#EB00;
    D_9 : word := W#16#60;
    D_10 : word := W#16#0;
    D_11 : word := W#16#1E1;
    D_12 : word := W#16#140;
    D_13 : word := W#16#0;
    D_14 : word := W#16#140;
    D_15 : word := W#16#0;
    D_16 : word := W#16#8000;
    D_17 : word := W#16#0;
    D_18 : word := W#16#0;
    D_19 : word := W#16#0;
    D_20 : word := W#16#1;
    D_21 : word := W#16#0;
    D_22 : word := W#16#8000;
    D_23 : word := W#16#0;
    D_24 : word := W#16#0;
    D_25 : word := W#16#0;
    D_26 : word := W#16#0;
    D_27 : word := W#16#0;
    D_28 : word := W#16#0;
    D_29 : word := W#16#0;
    D_30 : word := W#16#0;
    D_31 : word := W#16#0;
    D_32 : word := W#16#0;
    D_33 : word := W#16#0;
    D_34 : word := W#16#0;
    D_35 : word := W#16#0;
    D_36 : word := W#16#8085;
    D_37 : word := W#16#3E00;
    D_38 : word := W#16#60;
    D_39 : word := W#16#0;
    D_40 : word := W#16#8000;
    D_41 : word := W#16#0;
    D_42 : word := W#16#0;
    D_43 : word := W#16#0;
    D_44 : word := W#16#140;
    D_45 : word := W#16#100;
    D_46 : word := W#16#140;
    D_47 : word := W#16#0;
    D_48 : word := W#16#7FFF;
  END_STRUCT
BEGIN

END_DATA_BLOCK

DATA_BLOCK DB 212


STRUCT
    D_0 : word := W#16#0;
    D_1 : word := W#16#FD99;
    D_2 : word := W#16#999A;
    D_3 : word := W#16#140;
    D_4 : word := W#16#0;
    D_5 : word := W#16#FC6A;
    D_6 : word := W#16#1C00;
    D_7 : word := W#16#FC51;
    D_8 : word := W#16#EB00;
    D_9 : word := W#16#E9AE;
    D_10 : word := W#16#1500;
    D_11 : word := W#16#1E0;
    D_12 : word := W#16#FF66;
    D_13 : word := W#16#6600;
    D_14 : word := W#16#140;
    D_15 : word := W#16#0;
    D_16 : word := W#16#8000;
    D_17 : word := W#16#0;
    D_18 : word := W#16#0;
    D_19 : word := W#16#0;
    D_20 : word := W#16#300;
    D_21 : word := W#16#0;
    D_22 : word := W#16#FAB0;
    D_23 : word := W#16#0;
    D_24 : word := W#16#0;
    D_25 : word := W#16#0;
    D_26 : word := W#16#0;
    D_27 : word := W#16#0;
    D_28 : word := W#16#0;
    D_29 : word := W#16#0;
    D_30 : word := W#16#0;
    D_31 : word := W#16#0;
    D_32 : word := W#16#0;
    D_33 : word := W#16#0;
    D_34 : word := W#16#0;
    D_35 : word := W#16#0;
    D_36 : word := W#16#0;
    D_37 : word := W#16#0;
    D_38 : word := W#16#0;
    D_39 : word := W#16#0;
    D_40 : word := W#16#0;
    D_41 : word := W#16#0;
    D_42 : word := W#16#0;
    D_43 : word := W#16#0;
    D_44 : word := W#16#FF66;
    D_45 : word := W#16#6600;
    D_46 : word := W#16#FF66;
    D_47 : word := W#16#6600;
    D_48 : word := W#16#3333;
  END_STRUCT
BEGIN

END_DATA_BLOCK

DATA_BLOCK DB 213


STRUCT
    D_0 : word := W#16#0;
    D_1 : word := W#16#376;
    D_2 : word := W#16#0;
    D_3 : word := W#16#140;
    D_4 : word := W#16#0;
    D_5 : word := W#16#FA5B;
    D_6 : word := W#16#400;
    D_7 : word := W#16#55A;
    D_8 : word := W#16#0;
    D_9 : word := W#16#55;
    D_10 : word := W#16#5400;
    D_11 : word := W#16#1E0;
    D_12 : word := W#16#8000;
    D_13 : word := W#16#0;
    D_14 : word := W#16#140;
    D_15 : word := W#16#0;
    D_16 : word := W#16#8000;
    D_17 : word := W#16#0;
    D_18 : word := W#16#0;
    D_19 : word := W#16#0;
    D_20 : word := W#16#300;
    D_21 : word := W#16#0;
    D_22 : word := W#16#153;
    D_23 : word := W#16#1500;
    D_24 : word := W#16#0;
    D_25 : word := W#16#0;
    D_26 : word := W#16#0;
    D_27 : word := W#16#0;
    D_28 : word := W#16#0;
    D_29 : word := W#16#0;
    D_30 : word := W#16#0;
    D_31 : word := W#16#0;
    D_32 : word := W#16#0;
    D_33 : word := W#16#0;
    D_34 : word := W#16#0;
    D_35 : word := W#16#0;
    D_36 : word := W#16#0;
    D_37 : word := W#16#0;
    D_38 : word := W#16#0;
    D_39 : word := W#16#0;
    D_40 : word := W#16#0;
    D_41 : word := W#16#0;
    D_42 : word := W#16#0;
    D_43 : word := W#16#0;
    D_44 : word := W#16#0;
    D_45 : word := W#16#0;
    D_46 : word := W#16#0;
    D_47 : word := W#16#0;
    D_48 : word := W#16#0;
  END_STRUCT
BEGIN

END_DATA_BLOCK

DATA_BLOCK DB 214


STRUCT
    D_0 : word := W#16#0;
    D_1 : word := W#16#376;
    D_2 : word := W#16#0;
    D_3 : word := W#16#140;
    D_4 : word := W#16#0;
    D_5 : word := W#16#FA5B;
    D_6 : word := W#16#400;
    D_7 : word := W#16#55A;
    D_8 : word := W#16#0;
    D_9 : word := W#16#40;
    D_10 : word := W#16#0;
    D_11 : word := W#16#1E0;
    D_12 : word := W#16#8000;
    D_13 : word := W#16#0;
    D_14 : word := W#16#140;
    D_15 : word := W#16#0;
    D_16 : word := W#16#8000;
    D_17 : word := W#16#0;
    D_18 : word := W#16#0;
    D_19 : word := W#16#0;
    D_20 : word := W#16#300;
    D_21 : word := W#16#0;
    D_22 : word := W#16#6E;
    D_23 : word := W#16#B400;
    D_24 : word := W#16#0;
    D_25 : word := W#16#0;
    D_26 : word := W#16#0;
    D_27 : word := W#16#0;
    D_28 : word := W#16#0;
    D_29 : word := W#16#0;
    D_30 : word := W#16#0;
    D_31 : word := W#16#0;
    D_32 : word := W#16#0;
    D_33 : word := W#16#0;
    D_34 : word := W#16#0;
    D_35 : word := W#16#0;
    D_36 : word := W#16#0;
    D_37 : word := W#16#0;
    D_38 : word := W#16#0;
    D_39 : word := W#16#0;
    D_40 : word := W#16#0;
    D_41 : word := W#16#0;
    D_42 : word := W#16#0;
    D_43 : word := W#16#0;
    D_44 : word := W#16#0;
    D_45 : word := W#16#0;
    D_46 : word := W#16#0;
    D_47 : word := W#16#0;
    D_48 : word := W#16#0;
  END_STRUCT
BEGIN

END_DATA_BLOCK

DATA_BLOCK DB 215


STRUCT
    D_0 : word := W#16#0;
    D_1 : word := W#16#376;
    D_2 : word := W#16#0;
    D_3 : word := W#16#140;
    D_4 : word := W#16#0;
    D_5 : word := W#16#FA5B;
    D_6 : word := W#16#400;
    D_7 : word := W#16#55A;
    D_8 : word := W#16#0;
    D_9 : word := W#16#FF7F;
    D_10 : word := W#16#FA00;
    D_11 : word := W#16#1E1;
    D_12 : word := W#16#140;
    D_13 : word := W#16#0;
    D_14 : word := W#16#140;
    D_15 : word := W#16#0;
    D_16 : word := W#16#8000;
    D_17 : word := W#16#0;
    D_18 : word := W#16#0;
    D_19 : word := W#16#0;
    D_20 : word := W#16#2;
    D_21 : word := W#16#0;
    D_22 : word := W#16#160;
    D_23 : word := W#16#B400;
    D_24 : word := W#16#0;
    D_25 : word := W#16#0;
    D_26 : word := W#16#0;
    D_27 : word := W#16#0;
    D_28 : word := W#16#0;
    D_29 : word := W#16#0;
    D_30 : word := W#16#0;
    D_31 : word := W#16#0;
    D_32 : word := W#16#0;
    D_33 : word := W#16#0;
    D_34 : word := W#16#0;
    D_35 : word := W#16#0;
    D_36 : word := W#16#F0BC;
    D_37 : word := W#16#8000;
    D_38 : word := W#16#1BF;
    D_39 : word := W#16#4B00;
    D_40 : word := W#16#8000;
    D_41 : word := W#16#0;
    D_42 : word := W#16#0;
    D_43 : word := W#16#0;
    D_44 : word := W#16#4BE;
    D_45 : word := W#16#3700;
    D_46 : word := W#16#8000;
    D_47 : word := W#16#0;
    D_48 : word := W#16#0;
  END_STRUCT
BEGIN

END_DATA_BLOCK

DATA_BLOCK DB 216


STRUCT
    D_0 : word := W#16#0;
    D_1 : word := W#16#376;
    D_2 : word := W#16#0;
    D_3 : word := W#16#140;
    D_4 : word := W#16#0;
    D_5 : word := W#16#FC44;
    D_6 : word := W#16#FC00;
    D_7 : word := W#16#36E;
    D_8 : word := W#16#0;
    D_9 : word := W#16#4A;
    D_10 : word := W#16#3C00;
    D_11 : word := W#16#1E0;
    D_12 : word := W#16#8000;
    D_13 : word := W#16#0;
    D_14 : word := W#16#140;
    D_15 : word := W#16#0;
    D_16 : word := W#16#8000;
    D_17 : word := W#16#0;
    D_18 : word := W#16#0;
    D_19 : word := W#16#0;
    D_20 : word := W#16#300;
    D_21 : word := W#16#0;
    D_22 : word := W#16#F540;
    D_23 : word := W#16#0;
    D_24 : word := W#16#0;
    D_25 : word := W#16#0;
    D_26 : word := W#16#0;
    D_27 : word := W#16#0;
    D_28 : word := W#16#0;
    D_29 : word := W#16#0;
    D_30 : word := W#16#0;
    D_31 : word := W#16#0;
    D_32 : word := W#16#0;
    D_33 : word := W#16#0;
    D_34 : word := W#16#0;
    D_35 : word := W#16#0;
    D_36 : word := W#16#0;
    D_37 : word := W#16#0;
    D_38 : word := W#16#0;
    D_39 : word := W#16#0;
    D_40 : word := W#16#0;
    D_41 : word := W#16#0;
    D_42 : word := W#16#0;
    D_43 : word := W#16#0;
    D_44 : word := W#16#0;
    D_45 : word := W#16#0;
    D_46 : word := W#16#0;
    D_47 : word := W#16#0;
    D_48 : word := W#16#0;
  END_STRUCT
BEGIN

END_DATA_BLOCK

DATA_BLOCK DB 217


STRUCT
    D_0 : word := W#16#0;
    D_1 : word := W#16#376;
    D_2 : word := W#16#0;
    D_3 : word := W#16#140;
    D_4 : word := W#16#0;
    D_5 : word := W#16#FC44;
    D_6 : word := W#16#FB00;
    D_7 : word := W#16#47D;
    D_8 : word := W#16#0;
    D_9 : word := W#16#4C;
    D_10 : word := W#16#CC00;
    D_11 : word := W#16#1E0;
    D_12 : word := W#16#8000;
    D_13 : word := W#16#0;
    D_14 : word := W#16#140;
    D_15 : word := W#16#0;
    D_16 : word := W#16#8000;
    D_17 : word := W#16#0;
    D_18 : word := W#16#0;
    D_19 : word := W#16#0;
    D_20 : word := W#16#300;
    D_21 : word := W#16#0;
    D_22 : word := W#16#FB65;
    D_23 : word := W#16#0;
    D_24 : word := W#16#0;
    D_25 : word := W#16#0;
    D_26 : word := W#16#0;
    D_27 : word := W#16#0;
    D_28 : word := W#16#0;
    D_29 : word := W#16#0;
    D_30 : word := W#16#0;
    D_31 : word := W#16#0;
    D_32 : word := W#16#0;
    D_33 : word := W#16#0;
    D_34 : word := W#16#0;
    D_35 : word := W#16#0;
    D_36 : word := W#16#0;
    D_37 : word := W#16#0;
    D_38 : word := W#16#0;
    D_39 : word := W#16#0;
    D_40 : word := W#16#0;
    D_41 : word := W#16#0;
    D_42 : word := W#16#0;
    D_43 : word := W#16#0;
    D_44 : word := W#16#0;
    D_45 : word := W#16#0;
    D_46 : word := W#16#0;
    D_47 : word := W#16#0;
    D_48 : word := W#16#0;
  END_STRUCT
BEGIN

END_DATA_BLOCK

DATA_BLOCK DB 218


STRUCT
    D_0 : word := W#16#0;
    D_1 : word := W#16#3AD;
    D_2 : word := W#16#1EB9;
    D_3 : word := W#16#140;
    D_4 : word := W#16#0;
    D_5 : word := W#16#FC4A;
    D_6 : word := W#16#7800;
    D_7 : word := W#16#346;
    D_8 : word := W#16#0;
    D_9 : word := W#16#4E;
    D_10 : word := W#16#B800;
    D_11 : word := W#16#1E0;
    D_12 : word := W#16#8000;
    D_13 : word := W#16#0;
    D_14 : word := W#16#140;
    D_15 : word := W#16#0;
    D_16 : word := W#16#8000;
    D_17 : word := W#16#0;
    D_18 : word := W#16#0;
    D_19 : word := W#16#0;
    D_20 : word := W#16#300;
    D_21 : word := W#16#0;
    D_22 : word := W#16#141;
    D_23 : word := W#16#F00;
    D_24 : word := W#16#0;
    D_25 : word := W#16#0;
    D_26 : word := W#16#0;
    D_27 : word := W#16#0;
    D_28 : word := W#16#0;
    D_29 : word := W#16#0;
    D_30 : word := W#16#0;
    D_31 : word := W#16#0;
    D_32 : word := W#16#0;
    D_33 : word := W#16#0;
    D_34 : word := W#16#0;
    D_35 : word := W#16#0;
    D_36 : word := W#16#0;
    D_37 : word := W#16#0;
    D_38 : word := W#16#0;
    D_39 : word := W#16#0;
    D_40 : word := W#16#0;
    D_41 : word := W#16#0;
    D_42 : word := W#16#0;
    D_43 : word := W#16#0;
    D_44 : word := W#16#0;
    D_45 : word := W#16#0;
    D_46 : word := W#16#0;
    D_47 : word := W#16#0;
    D_48 : word := W#16#0;
  END_STRUCT
BEGIN

END_DATA_BLOCK

DATA_BLOCK DB 219


STRUCT
    D_0 : word := W#16#0;
    D_1 : word := W#16#2B4;
    D_2 : word := W#16#E14A;
    D_3 : word := W#16#140;
    D_4 : word := W#16#0;
    D_5 : word := W#16#FF51;
    D_6 : word := W#16#EC00;
    D_7 : word := W#16#152;
    D_8 : word := W#16#3200;
    D_9 : word := W#16#FE4C;
    D_10 : word := W#16#CC00;
    D_11 : word := W#16#1E1;
    D_12 : word := W#16#FE66;
    D_13 : word := W#16#6600;
    D_14 : word := W#16#140;
    D_15 : word := W#16#0;
    D_16 : word := W#16#8000;
    D_17 : word := W#16#0;
    D_18 : word := W#16#0;
    D_19 : word := W#16#0;
    D_20 : word := W#16#0;
    D_21 : word := W#16#0;
    D_22 : word := W#16#0;
    D_23 : word := W#16#0;
    D_24 : word := W#16#0;
    D_25 : word := W#16#0;
    D_26 : word := W#16#0;
    D_27 : word := W#16#0;
    D_28 : word := W#16#0;
    D_29 : word := W#16#0;
    D_30 : word := W#16#0;
    D_31 : word := W#16#0;
    D_32 : word := W#16#0;
    D_33 : word := W#16#0;
    D_34 : word := W#16#0;
    D_35 : word := W#16#0;
    D_36 : word := W#16#0;
    D_37 : word := W#16#0;
    D_38 : word := W#16#0;
    D_39 : word := W#16#0;
    D_40 : word := W#16#0;
    D_41 : word := W#16#0;
    D_42 : word := W#16#0;
    D_43 : word := W#16#0;
    D_44 : word := W#16#0;
    D_45 : word := W#16#0;
    D_46 : word := W#16#0;
    D_47 : word := W#16#0;
    D_48 : word := W#16#7FFF;
  END_STRUCT
BEGIN

END_DATA_BLOCK

DATA_BLOCK DB 220


STRUCT
    D_0 : word := W#16#0;
    D_1 : word := W#16#29C;
    D_2 : word := W#16#B733;
    D_3 : word := W#16#140;
    D_4 : word := W#16#0;
    D_5 : word := W#16#FD51;
    D_6 : word := W#16#EC00;
    D_7 : word := W#16#350;
    D_8 : word := W#16#3200;
    D_9 : word := W#16#FE47;
    D_10 : word := W#16#AE00;
    D_11 : word := W#16#1E0;
    D_12 : word := W#16#FD66;
    D_13 : word := W#16#6600;
    D_14 : word := W#16#140;
    D_15 : word := W#16#0;
    D_16 : word := W#16#8000;
    D_17 : word := W#16#0;
    D_18 : word := W#16#0;
    D_19 : word := W#16#0;
    D_20 : word := W#16#300;
    D_21 : word := W#16#0;
    D_22 : word := W#16#FE65;
    D_23 : word := W#16#0;
    D_24 : word := W#16#0;
    D_25 : word := W#16#0;
    D_26 : word := W#16#0;
    D_27 : word := W#16#0;
    D_28 : word := W#16#0;
    D_29 : word := W#16#0;
    D_30 : word := W#16#0;
    D_31 : word := W#16#0;
    D_32 : word := W#16#0;
    D_33 : word := W#16#0;
    D_34 : word := W#16#0;
    D_35 : word := W#16#0;
    D_36 : word := W#16#0;
    D_37 : word := W#16#0;
    D_38 : word := W#16#0;
    D_39 : word := W#16#0;
    D_40 : word := W#16#0;
    D_41 : word := W#16#0;
    D_42 : word := W#16#0;
    D_43 : word := W#16#0;
    D_44 : word := W#16#FD66;
    D_45 : word := W#16#6600;
    D_46 : word := W#16#FD66;
    D_47 : word := W#16#6600;
    D_48 : word := W#16#CCC;
  END_STRUCT
BEGIN

END_DATA_BLOCK

DATA_BLOCK DB 221


STRUCT
    D_0 : word := W#16#0;
    D_1 : word := W#16#4A8;
    D_2 : word := W#16#0;
    D_3 : word := W#16#140;
    D_4 : word := W#16#0;
    D_5 : word := W#16#FA45;
    D_6 : word := W#16#B700;
    D_7 : word := W#16#564;
    D_8 : word := W#16#C00;
    D_9 : word := W#16#41;
    D_10 : word := W#16#4700;
    D_11 : word := W#16#1E1;
    D_12 : word := W#16#FD66;
    D_13 : word := W#16#6600;
    D_14 : word := W#16#140;
    D_15 : word := W#16#0;
    D_16 : word := W#16#8000;
    D_17 : word := W#16#0;
    D_18 : word := W#16#0;
    D_19 : word := W#16#0;
    D_20 : word := W#16#1;
    D_21 : word := W#16#0;
    D_22 : word := W#16#4B;
    D_23 : word := W#16#C000;
    D_24 : word := W#16#0;
    D_25 : word := W#16#0;
    D_26 : word := W#16#0;
    D_27 : word := W#16#0;
    D_28 : word := W#16#0;
    D_29 : word := W#16#0;
    D_30 : word := W#16#0;
    D_31 : word := W#16#0;
    D_32 : word := W#16#0;
    D_33 : word := W#16#0;
    D_34 : word := W#16#0;
    D_35 : word := W#16#0;
    D_36 : word := W#16#A767;
    D_37 : word := W#16#3000;
    D_38 : word := W#16#FDAC;
    D_39 : word := W#16#3800;
    D_40 : word := W#16#8000;
    D_41 : word := W#16#0;
    D_42 : word := W#16#0;
    D_43 : word := W#16#0;
    D_44 : word := W#16#243;
    D_45 : word := W#16#100;
    D_46 : word := W#16#140;
    D_47 : word := W#16#0;
    D_48 : word := W#16#7FFF;
  END_STRUCT
BEGIN

END_DATA_BLOCK

DATA_BLOCK DB 222


STRUCT
    D_0 : word := W#16#0;
    D_1 : word := W#16#180;
    D_2 : word := W#16#0;
    D_3 : word := W#16#140;
    D_4 : word := W#16#0;
    D_5 : word := W#16#166;
    D_6 : word := W#16#6600;
    D_7 : word := W#16#51;
    D_8 : word := W#16#3200;
    D_9 : word := W#16#FF5A;
    D_10 : word := W#16#E000;
    D_11 : word := W#16#1E0;
    D_12 : word := W#16#8000;
    D_13 : word := W#16#0;
    D_14 : word := W#16#140;
    D_15 : word := W#16#0;
    D_16 : word := W#16#8000;
    D_17 : word := W#16#0;
    D_18 : word := W#16#0;
    D_19 : word := W#16#0;
    D_20 : word := W#16#300;
    D_21 : word := W#16#0;
    D_22 : word := W#16#FE70;
    D_23 : word := W#16#8000;
    D_24 : word := W#16#0;
    D_25 : word := W#16#0;
    D_26 : word := W#16#0;
    D_27 : word := W#16#0;
    D_28 : word := W#16#0;
    D_29 : word := W#16#0;
    D_30 : word := W#16#0;
    D_31 : word := W#16#0;
    D_32 : word := W#16#0;
    D_33 : word := W#16#0;
    D_34 : word := W#16#0;
    D_35 : word := W#16#0;
    D_36 : word := W#16#0;
    D_37 : word := W#16#0;
    D_38 : word := W#16#0;
    D_39 : word := W#16#0;
    D_40 : word := W#16#0;
    D_41 : word := W#16#0;
    D_42 : word := W#16#0;
    D_43 : word := W#16#0;
    D_44 : word := W#16#0;
    D_45 : word := W#16#0;
    D_46 : word := W#16#0;
    D_47 : word := W#16#0;
    D_48 : word := W#16#0;
  END_STRUCT
BEGIN

END_DATA_BLOCK

DATA_BLOCK DB 223


STRUCT
    D_0 : word := W#16#0;
    D_1 : word := W#16#58B;
    D_2 : word := W#16#999B;
    D_3 : word := W#16#140;
    D_4 : word := W#16#0;
    D_5 : word := W#16#FC71;
    D_6 : word := W#16#C600;
    D_7 : word := W#16#FC51;
    D_8 : word := W#16#EB00;
    D_9 : word := W#16#FD4B;
    D_10 : word := W#16#1700;
    D_11 : word := W#16#1E1;
    D_12 : word := W#16#8000;
    D_13 : word := W#16#0;
    D_14 : word := W#16#140;
    D_15 : word := W#16#0;
    D_16 : word := W#16#8000;
    D_17 : word := W#16#0;
    D_18 : word := W#16#0;
    D_19 : word := W#16#0;
    D_20 : word := W#16#2;
    D_21 : word := W#16#0;
    D_22 : word := W#16#F9A8;
    D_23 : word := W#16#0;
    D_24 : word := W#16#0;
    D_25 : word := W#16#0;
    D_26 : word := W#16#0;
    D_27 : word := W#16#0;
    D_28 : word := W#16#0;
    D_29 : word := W#16#0;
    D_30 : word := W#16#0;
    D_31 : word := W#16#0;
    D_32 : word := W#16#0;
    D_33 : word := W#16#0;
    D_34 : word := W#16#0;
    D_35 : word := W#16#0;
    D_36 : word := W#16#80AC;
    D_37 : word := W#16#CC00;
    D_38 : word := W#16#FD50;
    D_39 : word := W#16#9700;
    D_40 : word := W#16#8000;
    D_41 : word := W#16#0;
    D_42 : word := W#16#0;
    D_43 : word := W#16#0;
    D_44 : word := W#16#2B4;
    D_45 : word := W#16#8900;
    D_46 : word := W#16#8000;
    D_47 : word := W#16#0;
    D_48 : word := W#16#0;
  END_STRUCT
BEGIN

END_DATA_BLOCK

DATA_BLOCK DB 224


STRUCT
    D_0 : word := W#16#0;
    D_1 : word := W#16#4C;
    D_2 : word := W#16#CC99;
    D_3 : word := W#16#140;
    D_4 : word := W#16#0;
    D_5 : word := W#16#FD66;
    D_6 : word := W#16#6600;
    D_7 : word := W#16#FB5A;
    D_8 : word := W#16#3900;
    D_9 : word := W#16#FE4C;
    D_10 : word := W#16#CC00;
    D_11 : word := W#16#1E1;
    D_12 : word := W#16#8000;
    D_13 : word := W#16#0;
    D_14 : word := W#16#140;
    D_15 : word := W#16#0;
    D_16 : word := W#16#8000;
    D_17 : word := W#16#0;
    D_18 : word := W#16#0;
    D_19 : word := W#16#0;
    D_20 : word := W#16#0;
    D_21 : word := W#16#0;
    D_22 : word := W#16#0;
    D_23 : word := W#16#0;
    D_24 : word := W#16#0;
    D_25 : word := W#16#0;
    D_26 : word := W#16#0;
    D_27 : word := W#16#0;
    D_28 : word := W#16#0;
    D_29 : word := W#16#0;
    D_30 : word := W#16#0;
    D_31 : word := W#16#0;
    D_32 : word := W#16#0;
    D_33 : word := W#16#0;
    D_34 : word := W#16#0;
    D_35 : word := W#16#0;
    D_36 : word := W#16#0;
    D_37 : word := W#16#0;
    D_38 : word := W#16#0;
    D_39 : word := W#16#0;
    D_40 : word := W#16#0;
    D_41 : word := W#16#0;
    D_42 : word := W#16#0;
    D_43 : word := W#16#0;
    D_44 : word := W#16#0;
    D_45 : word := W#16#0;
    D_46 : word := W#16#0;
    D_47 : word := W#16#0;
    D_48 : word := W#16#26EF;
  END_STRUCT
BEGIN

END_DATA_BLOCK

DATA_BLOCK DB 225


STRUCT
    D_0 : word := W#16#0;
    D_1 : word := W#16#FD51;
    D_2 : word := W#16#EB85;
    D_3 : word := W#16#140;
    D_4 : word := W#16#0;
    D_5 : word := W#16#166;
    D_6 : word := W#16#6600;
    D_7 : word := W#16#51;
    D_8 : word := W#16#3200;
    D_9 : word := W#16#FE7A;
    D_10 : word := W#16#E000;
    D_11 : word := W#16#1E0;
    D_12 : word := W#16#66;
    D_13 : word := W#16#6600;
    D_14 : word := W#16#140;
    D_15 : word := W#16#0;
    D_16 : word := W#16#8000;
    D_17 : word := W#16#0;
    D_18 : word := W#16#0;
    D_19 : word := W#16#0;
    D_20 : word := W#16#300;
    D_21 : word := W#16#0;
    D_22 : word := W#16#FF4B;
    D_23 : word := W#16#1E00;
    D_24 : word := W#16#0;
    D_25 : word := W#16#0;
    D_26 : word := W#16#0;
    D_27 : word := W#16#0;
    D_28 : word := W#16#0;
    D_29 : word := W#16#0;
    D_30 : word := W#16#0;
    D_31 : word := W#16#0;
    D_32 : word := W#16#0;
    D_33 : word := W#16#0;
    D_34 : word := W#16#0;
    D_35 : word := W#16#0;
    D_36 : word := W#16#0;
    D_37 : word := W#16#0;
    D_38 : word := W#16#0;
    D_39 : word := W#16#0;
    D_40 : word := W#16#0;
    D_41 : word := W#16#0;
    D_42 : word := W#16#0;
    D_43 : word := W#16#0;
    D_44 : word := W#16#66;
    D_45 : word := W#16#6600;
    D_46 : word := W#16#66;
    D_47 : word := W#16#6600;
    D_48 : word := W#16#6666;
  END_STRUCT
BEGIN

END_DATA_BLOCK

DATA_BLOCK DB 226


STRUCT
    D_0 : word := W#16#0;
    D_1 : word := W#16#FB46;
    D_2 : word := W#16#FB85;
    D_3 : word := W#16#140;
    D_4 : word := W#16#0;
    D_5 : word := W#16#FA52;
    D_6 : word := W#16#5500;
    D_7 : word := W#16#363;
    D_8 : word := W#16#FE00;
    D_9 : word := W#16#70;
    D_10 : word := W#16#0;
    D_11 : word := W#16#1E5;
    D_12 : word := W#16#8000;
    D_13 : word := W#16#0;
    D_14 : word := W#16#140;
    D_15 : word := W#16#0;
    D_16 : word := W#16#8000;
    D_17 : word := W#16#0;
    D_18 : word := W#16#0;
    D_19 : word := W#16#0;
    D_20 : word := W#16#4;
    D_21 : word := W#16#0;
    D_22 : word := W#16#FF60;
    D_23 : word := W#16#8000;
    D_24 : word := W#16#0;
    D_25 : word := W#16#0;
    D_26 : word := W#16#0;
    D_27 : word := W#16#0;
    D_28 : word := W#16#0;
    D_29 : word := W#16#0;
    D_30 : word := W#16#0;
    D_31 : word := W#16#0;
    D_32 : word := W#16#0;
    D_33 : word := W#16#0;
    D_34 : word := W#16#0;
    D_35 : word := W#16#0;
    D_36 : word := W#16#0;
    D_37 : word := W#16#0;
    D_38 : word := W#16#0;
    D_39 : word := W#16#0;
    D_40 : word := W#16#0;
    D_41 : word := W#16#0;
    D_42 : word := W#16#0;
    D_43 : word := W#16#0;
    D_44 : word := W#16#0;
    D_45 : word := W#16#0;
    D_46 : word := W#16#8000;
    D_47 : word := W#16#0;
    D_48 : word := W#16#0;
  END_STRUCT
BEGIN

END_DATA_BLOCK

DATA_BLOCK DB 227
  AUTHOR: _30057


STRUCT
    D_0 : word := W#16#0;
    D_1 : word := W#16#350;
    D_2 : word := W#16#0;
    D_3 : word := W#16#140;
    D_4 : word := W#16#0;
    D_5 : word := W#16#FE50;
    D_6 : word := W#16#5000;
    D_7 : word := W#16#FE40;
    D_8 : word := W#16#0;
    D_9 : word := W#16#47;
    D_10 : word := W#16#AE00;
    D_11 : word := W#16#1E1;
    D_12 : word := W#16#8000;
    D_13 : word := W#16#0;
    D_14 : word := W#16#140;
    D_15 : word := W#16#0;
    D_16 : word := W#16#8000;
    D_17 : word := W#16#0;
    D_18 : word := W#16#0;
    D_19 : word := W#16#0;
    D_20 : word := W#16#1;
    D_21 : word := W#16#0;
    D_22 : word := W#16#FF58;
    D_23 : word := W#16#9E00;
    D_24 : word := W#16#0;
    D_25 : word := W#16#0;
    D_26 : word := W#16#0;
    D_27 : word := W#16#0;
    D_28 : word := W#16#0;
    D_29 : word := W#16#0;
    D_30 : word := W#16#0;
    D_31 : word := W#16#0;
    D_32 : word := W#16#0;
    D_33 : word := W#16#0;
    D_34 : word := W#16#0;
    D_35 : word := W#16#0;
    D_36 : word := W#16#E470;
    D_37 : word := W#16#F800;
    D_38 : word := W#16#FE6D;
    D_39 : word := W#16#7C00;
    D_40 : word := W#16#8000;
    D_41 : word := W#16#0;
    D_42 : word := W#16#0;
    D_43 : word := W#16#0;
    D_44 : word := W#16#158;
    D_45 : word := W#16#7400;
    D_46 : word := W#16#140;
    D_47 : word := W#16#0;
    D_48 : word := W#16#7FFF;
  END_STRUCT
BEGIN

END_DATA_BLOCK

DATA_BLOCK DB 228
  AUTHOR: _30057


STRUCT
    D_0 : word := W#16#0;
    D_1 : word := W#16#153;
    D_2 : word := W#16#3333;
    D_3 : word := W#16#140;
    D_4 : word := W#16#0;
    D_5 : word := W#16#FE50;
    D_6 : word := W#16#5000;
    D_7 : word := W#16#40;
    D_8 : word := W#16#0;
    D_9 : word := W#16#5C;
    D_10 : word := W#16#2800;
    D_11 : word := W#16#1E5;
    D_12 : word := W#16#FF6B;
    D_13 : word := W#16#8400;
    D_14 : word := W#16#140;
    D_15 : word := W#16#0;
    D_16 : word := W#16#8000;
    D_17 : word := W#16#0;
    D_18 : word := W#16#0;
    D_19 : word := W#16#0;
    D_20 : word := W#16#0;
    D_21 : word := W#16#0;
    D_22 : word := W#16#0;
    D_23 : word := W#16#0;
    D_24 : word := W#16#0;
    D_25 : word := W#16#0;
    D_26 : word := W#16#0;
    D_27 : word := W#16#0;
    D_28 : word := W#16#0;
    D_29 : word := W#16#0;
    D_30 : word := W#16#0;
    D_31 : word := W#16#0;
    D_32 : word := W#16#0;
    D_33 : word := W#16#0;
    D_34 : word := W#16#0;
    D_35 : word := W#16#0;
    D_36 : word := W#16#0;
    D_37 : word := W#16#0;
    D_38 : word := W#16#0;
    D_39 : word := W#16#0;
    D_40 : word := W#16#0;
    D_41 : word := W#16#0;
    D_42 : word := W#16#0;
    D_43 : word := W#16#0;
    D_44 : word := W#16#0;
    D_45 : word := W#16#0;
    D_46 : word := W#16#0;
    D_47 : word := W#16#0;
    D_48 : word := W#16#0;
  END_STRUCT
BEGIN

END_DATA_BLOCK

DATA_BLOCK DB 256


STRUCT
    D_0 : word := W#16#4D41;
    D_1 : word := W#16#534B;
    D_2 : word := W#16#5830;
    D_3 : word := W#16#201;
    D_4 : word := W#16#3001;
    D_5 : word := W#16#402;
    D_6 : word := W#16#1000;
    D_7 : word := W#16#FA0;
    D_8 : word := W#16#EEEE;
  END_STRUCT
BEGIN

END_DATA_BLOCK
